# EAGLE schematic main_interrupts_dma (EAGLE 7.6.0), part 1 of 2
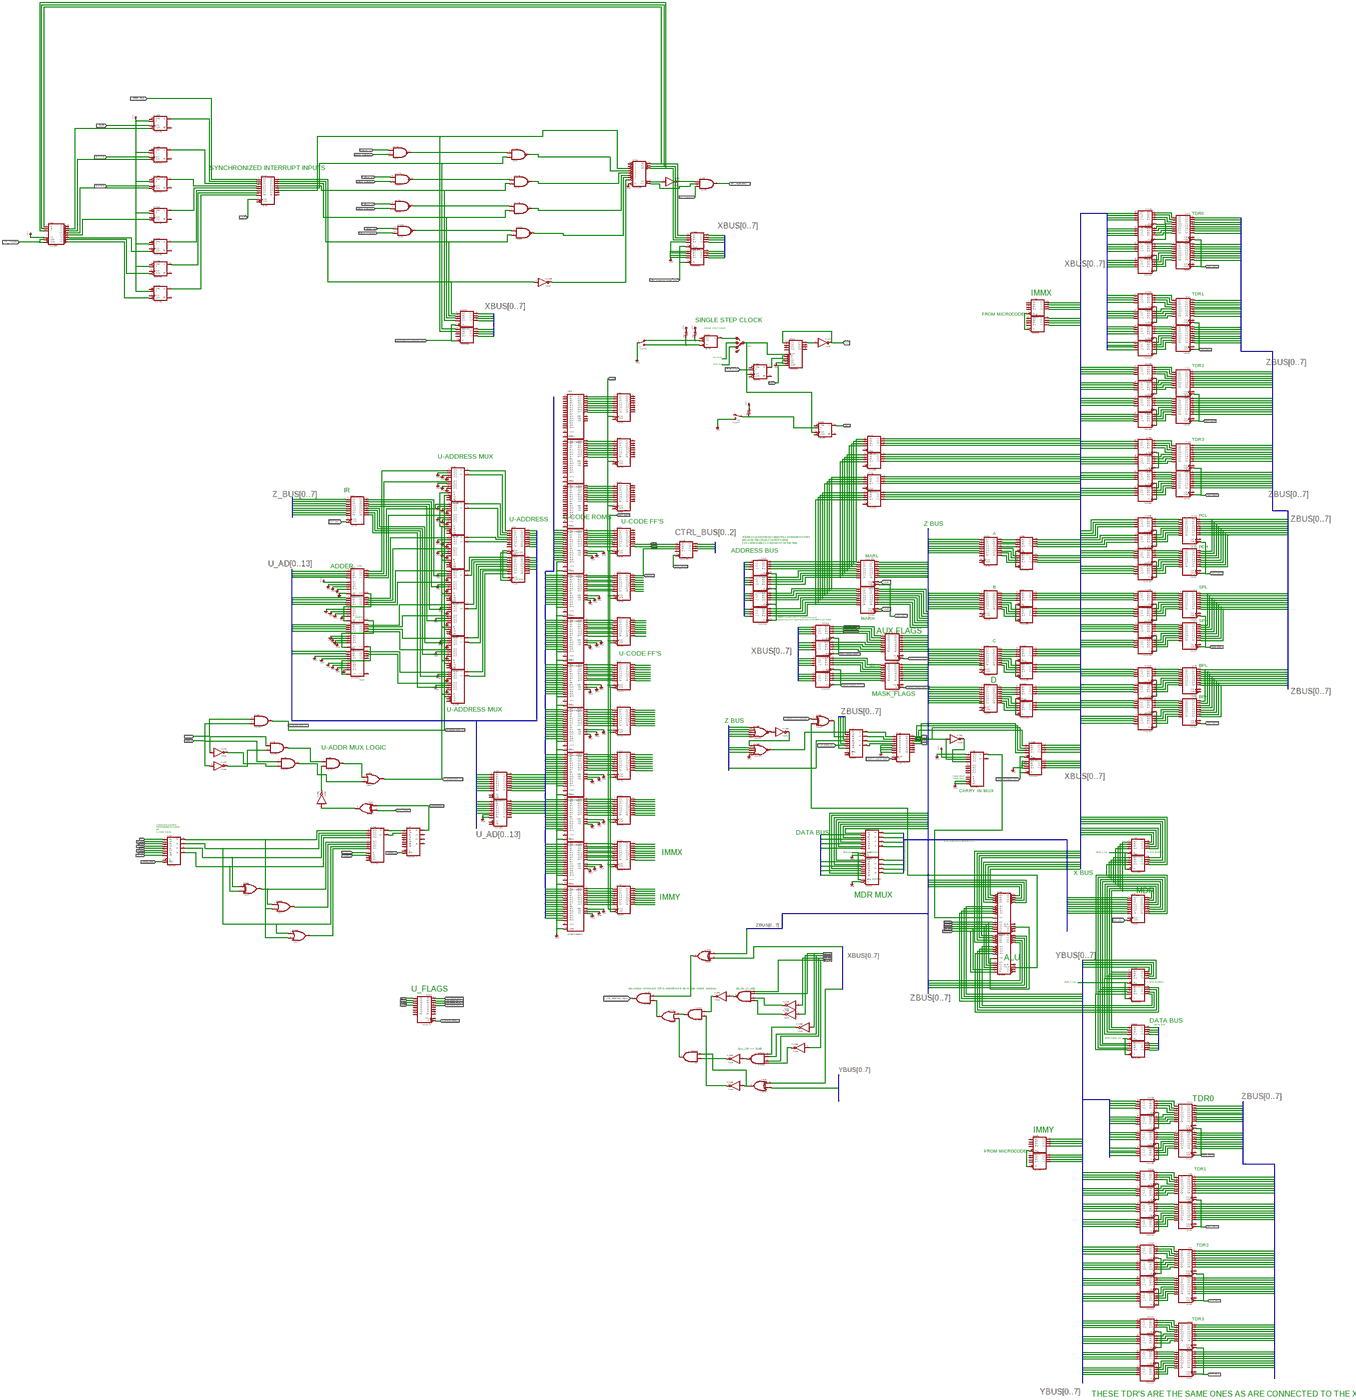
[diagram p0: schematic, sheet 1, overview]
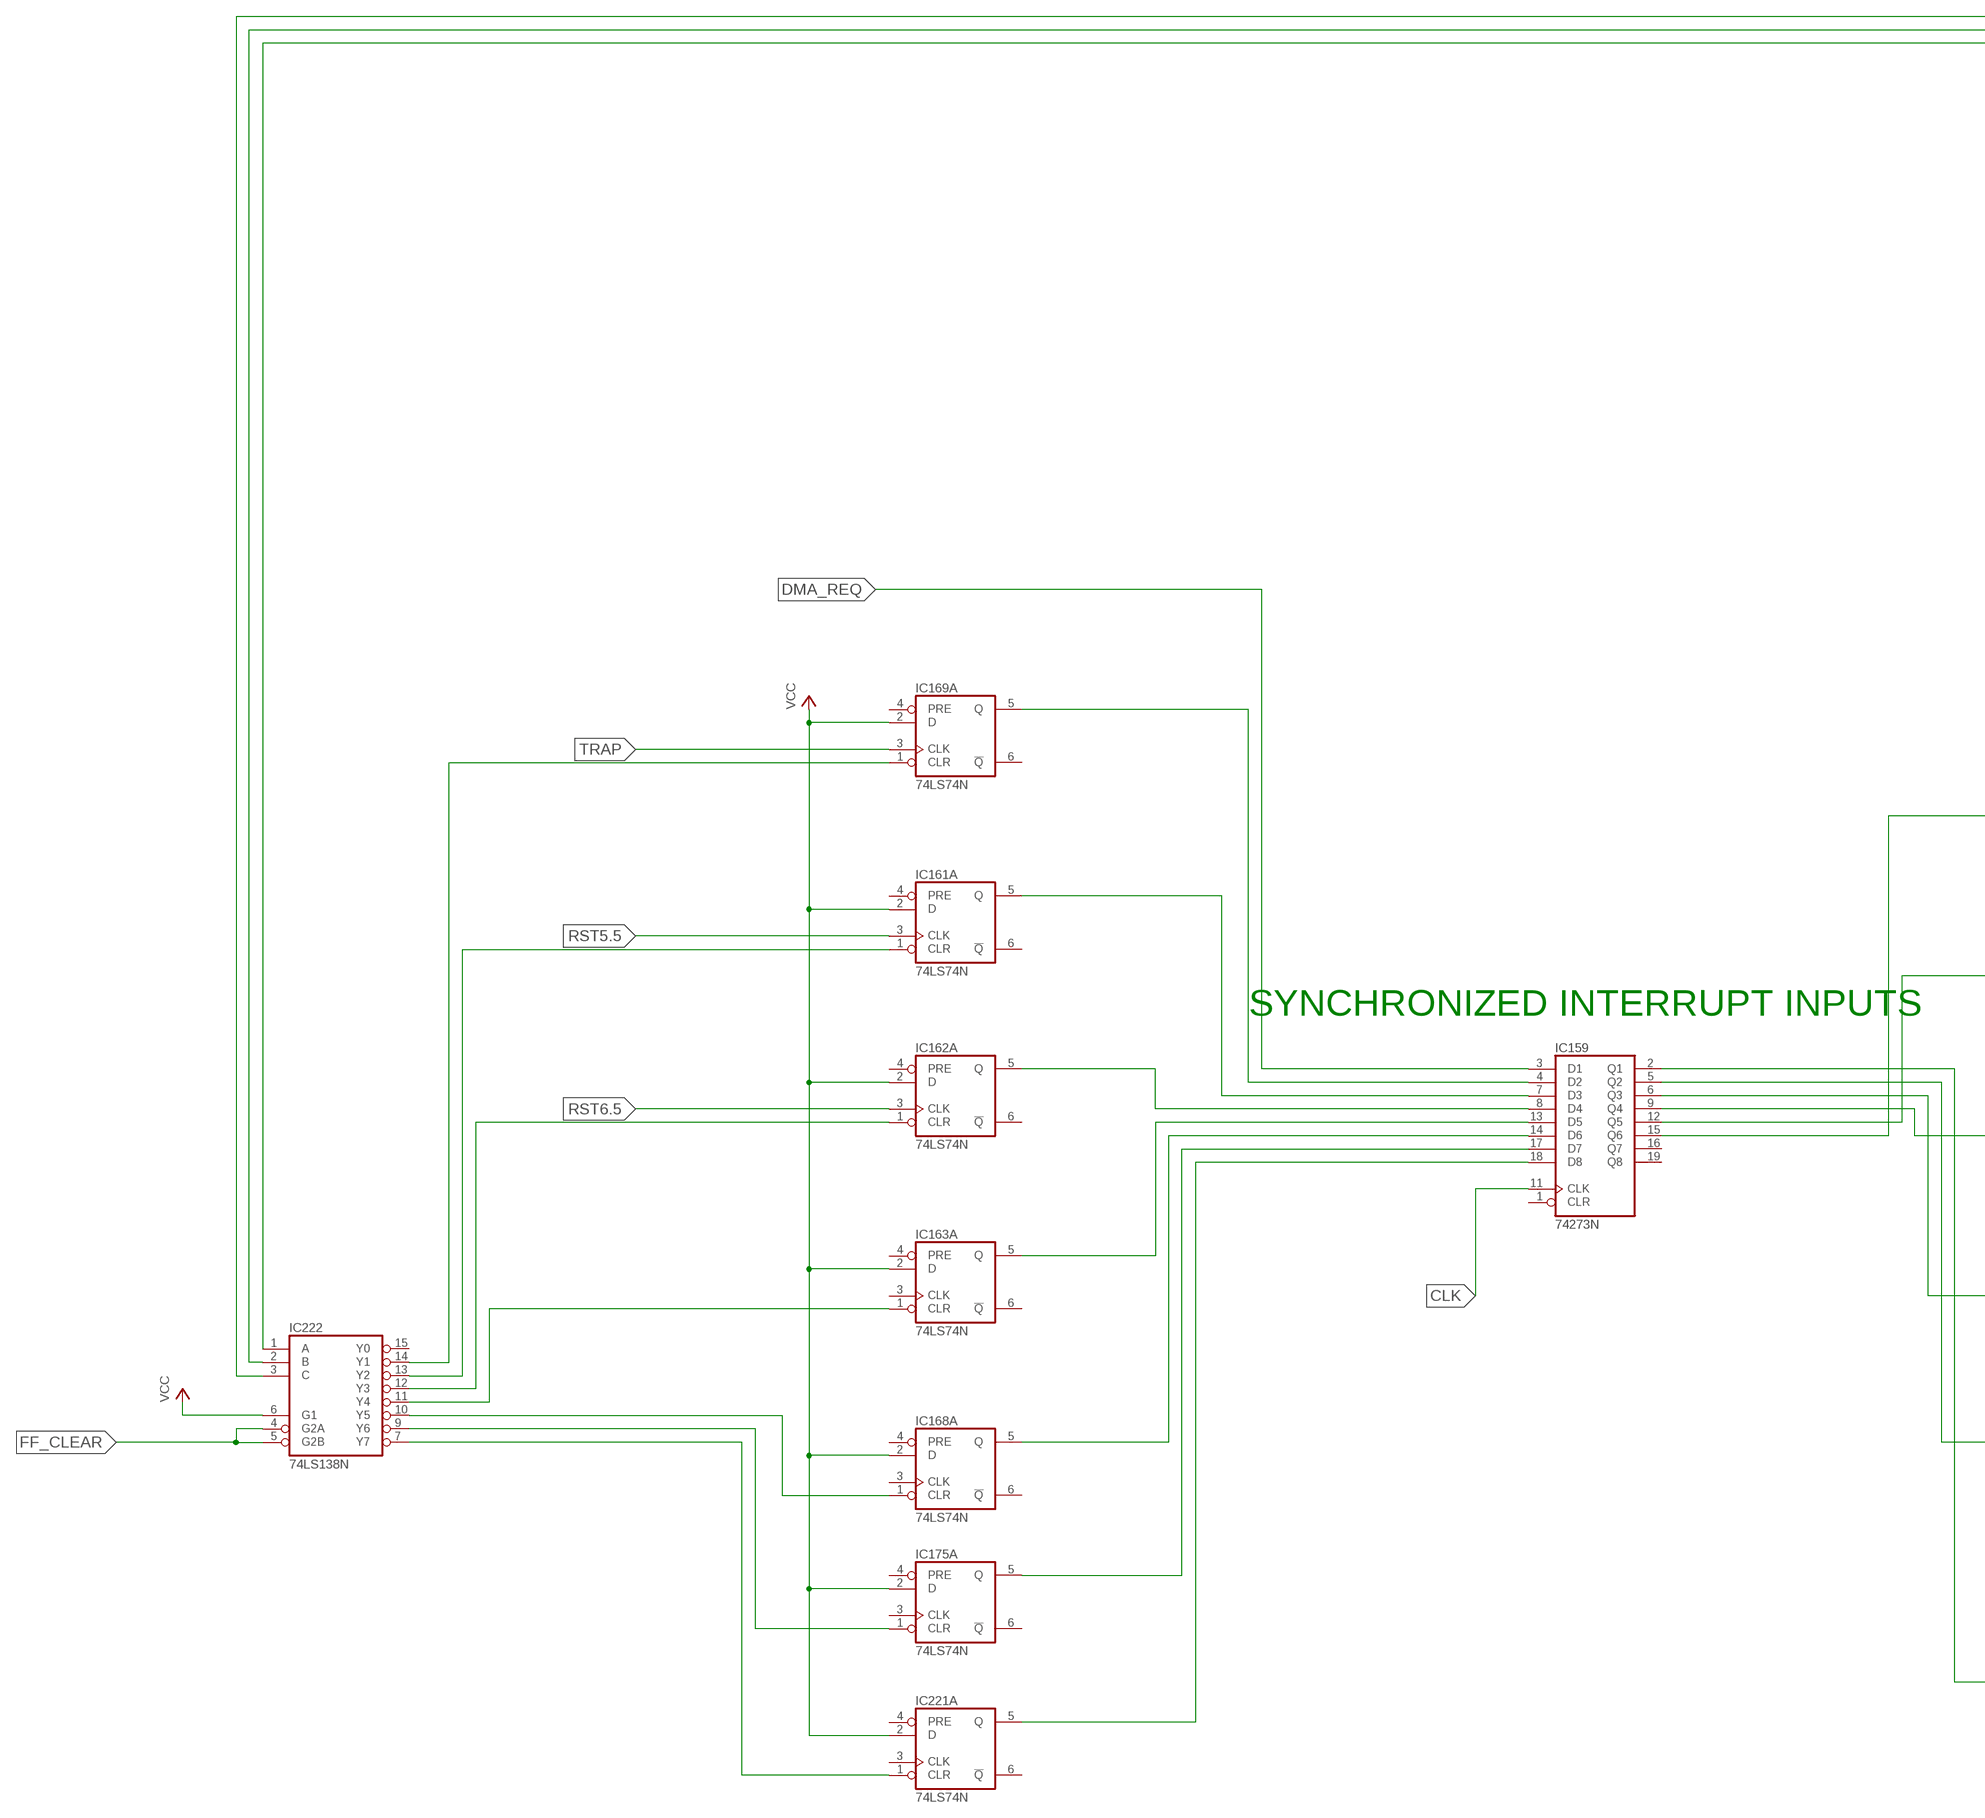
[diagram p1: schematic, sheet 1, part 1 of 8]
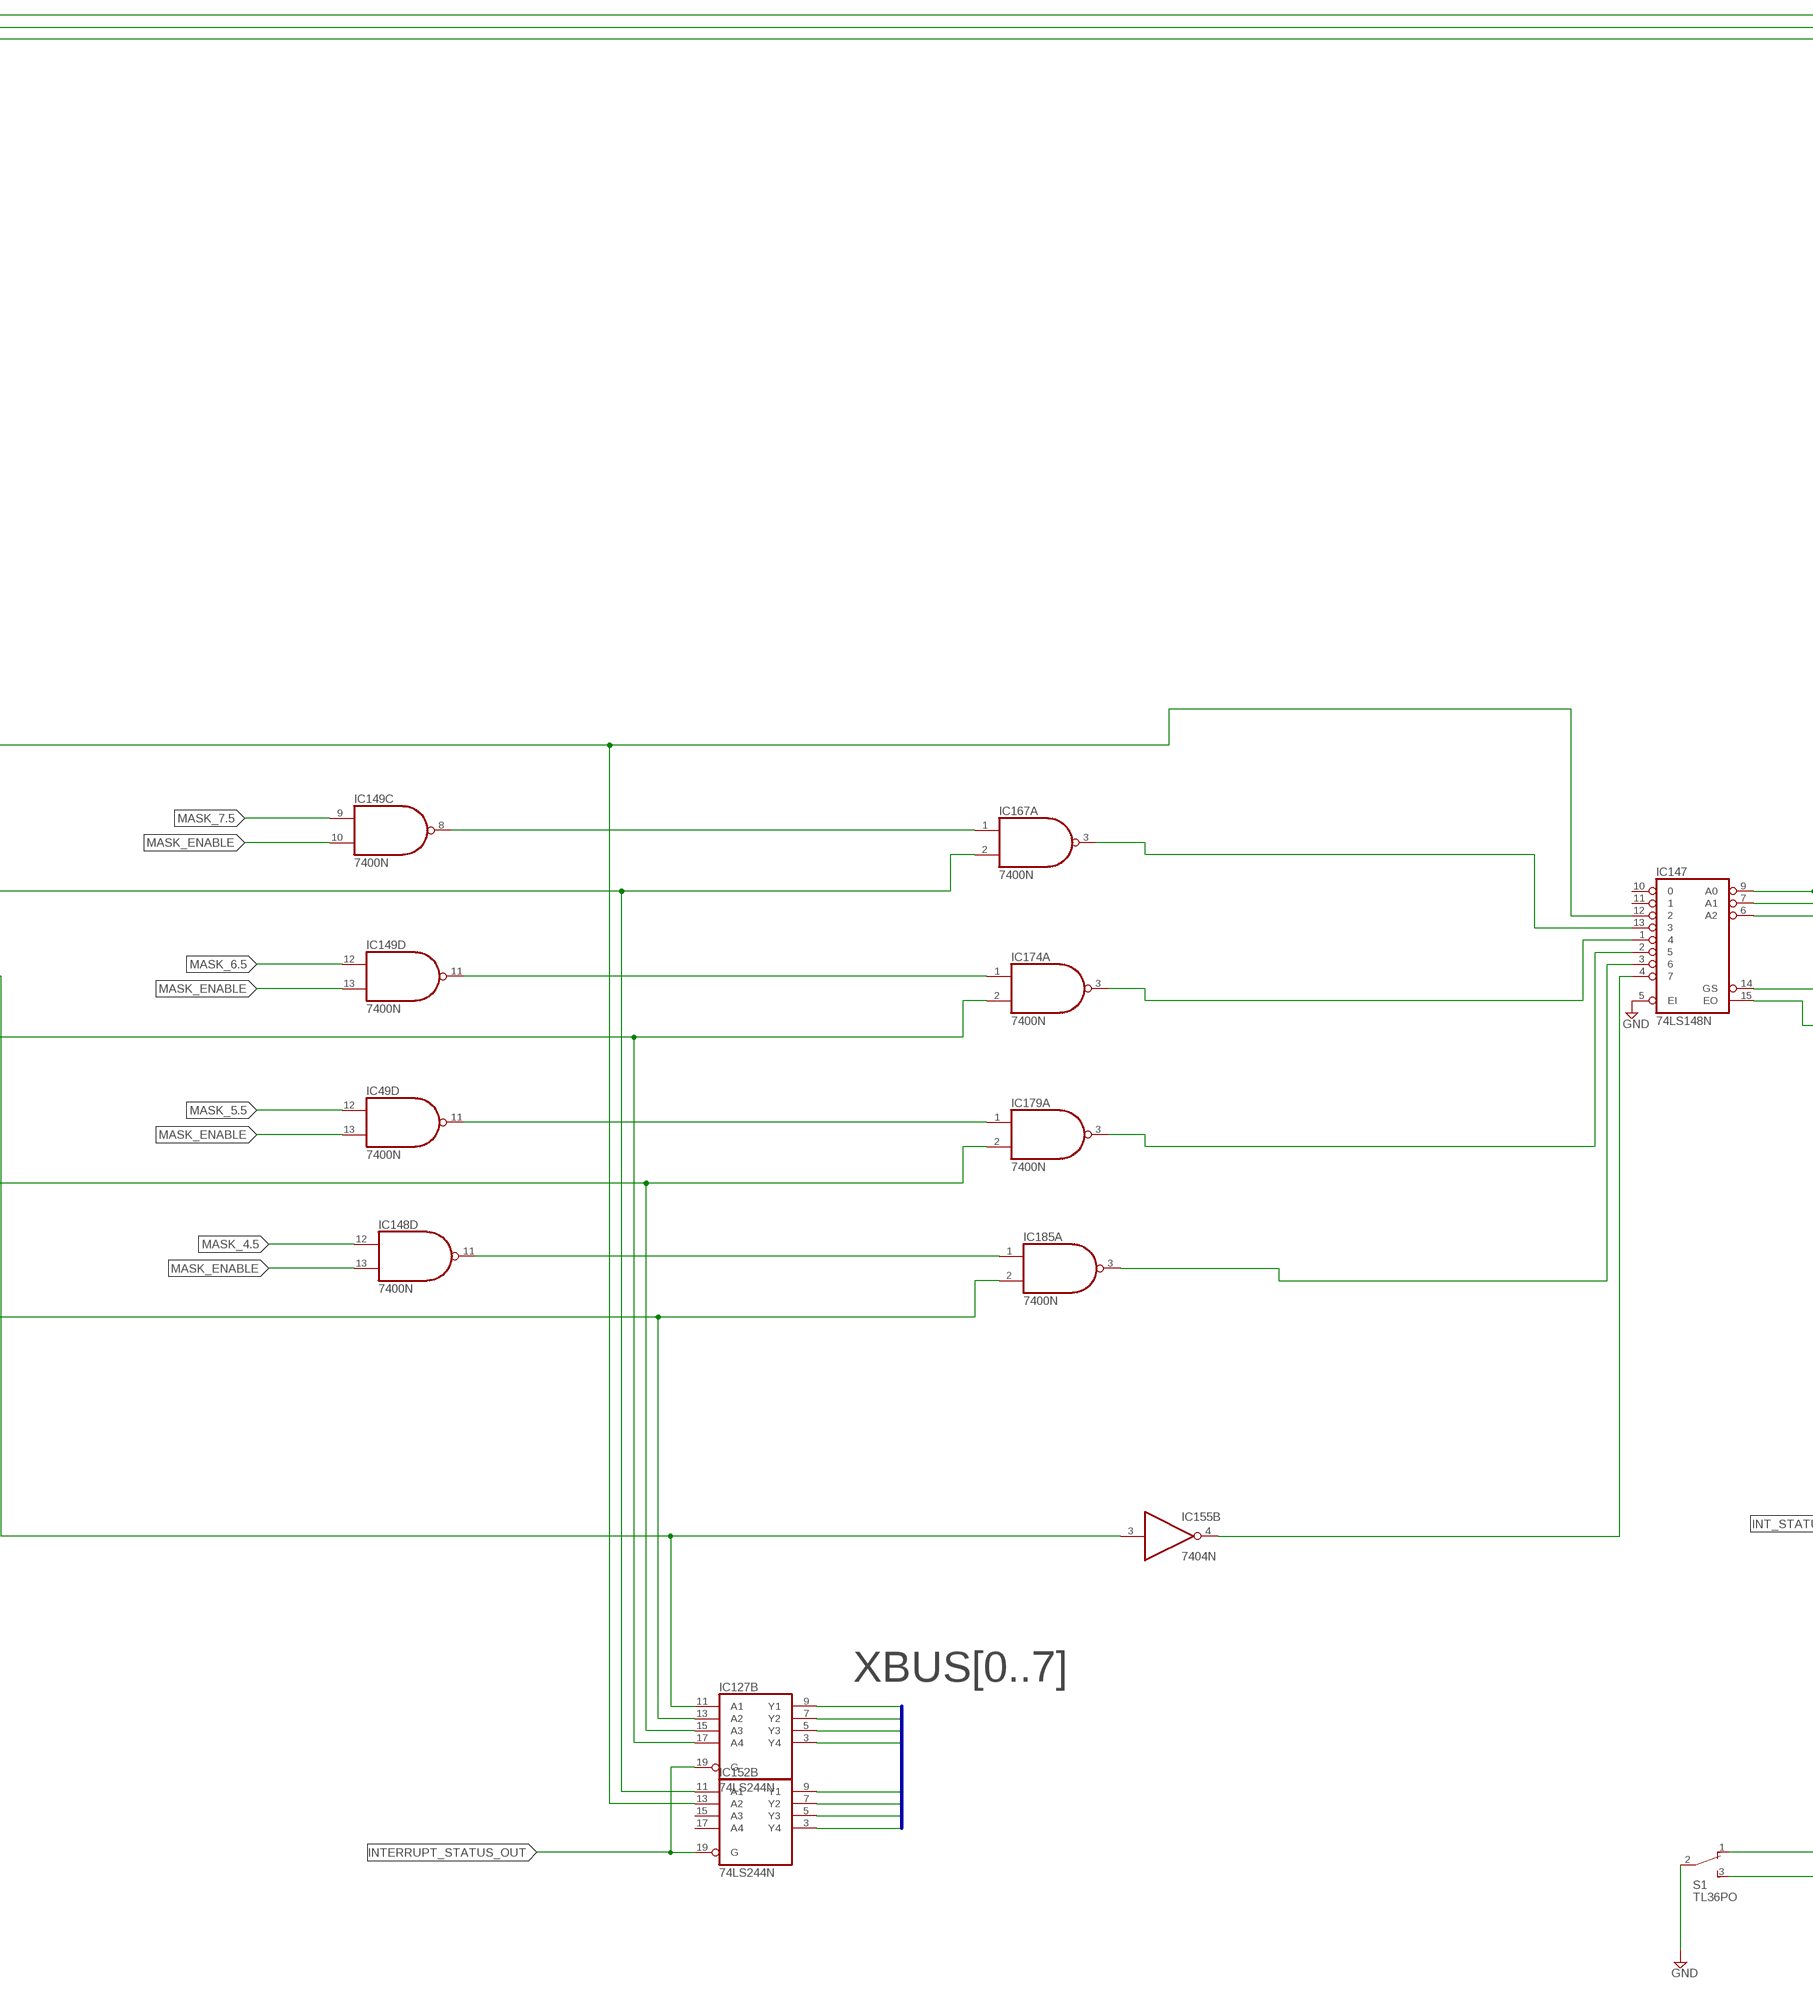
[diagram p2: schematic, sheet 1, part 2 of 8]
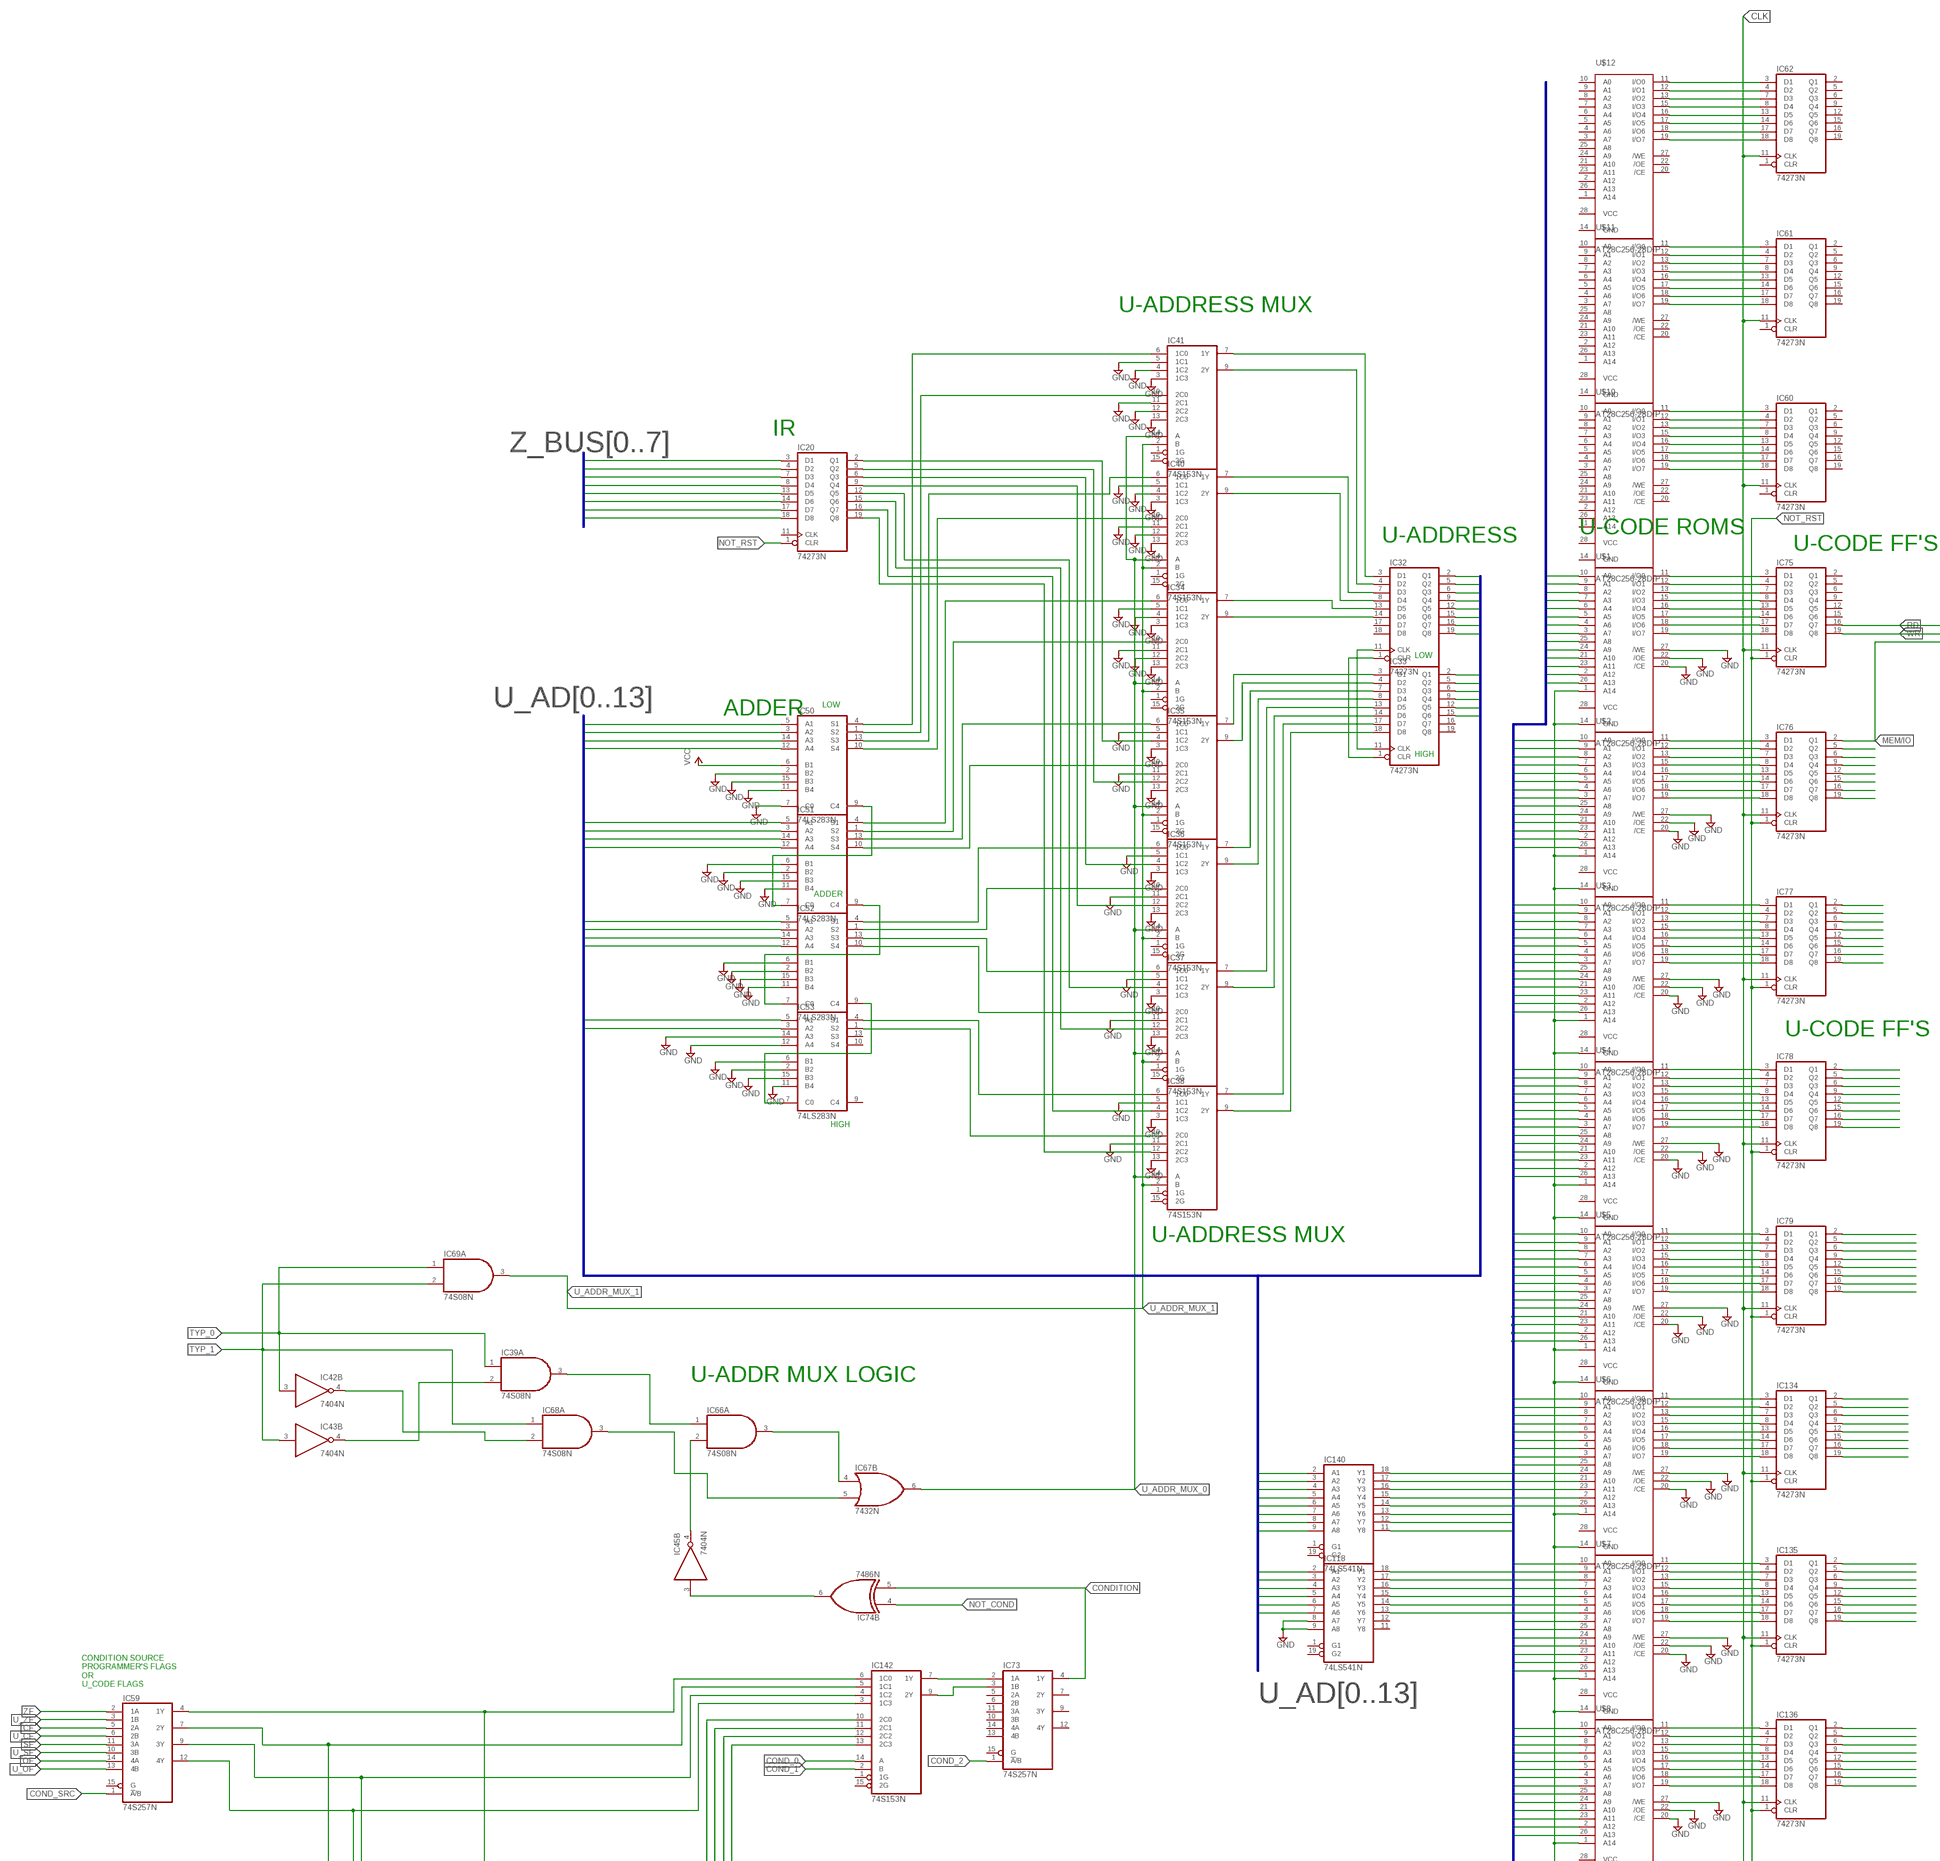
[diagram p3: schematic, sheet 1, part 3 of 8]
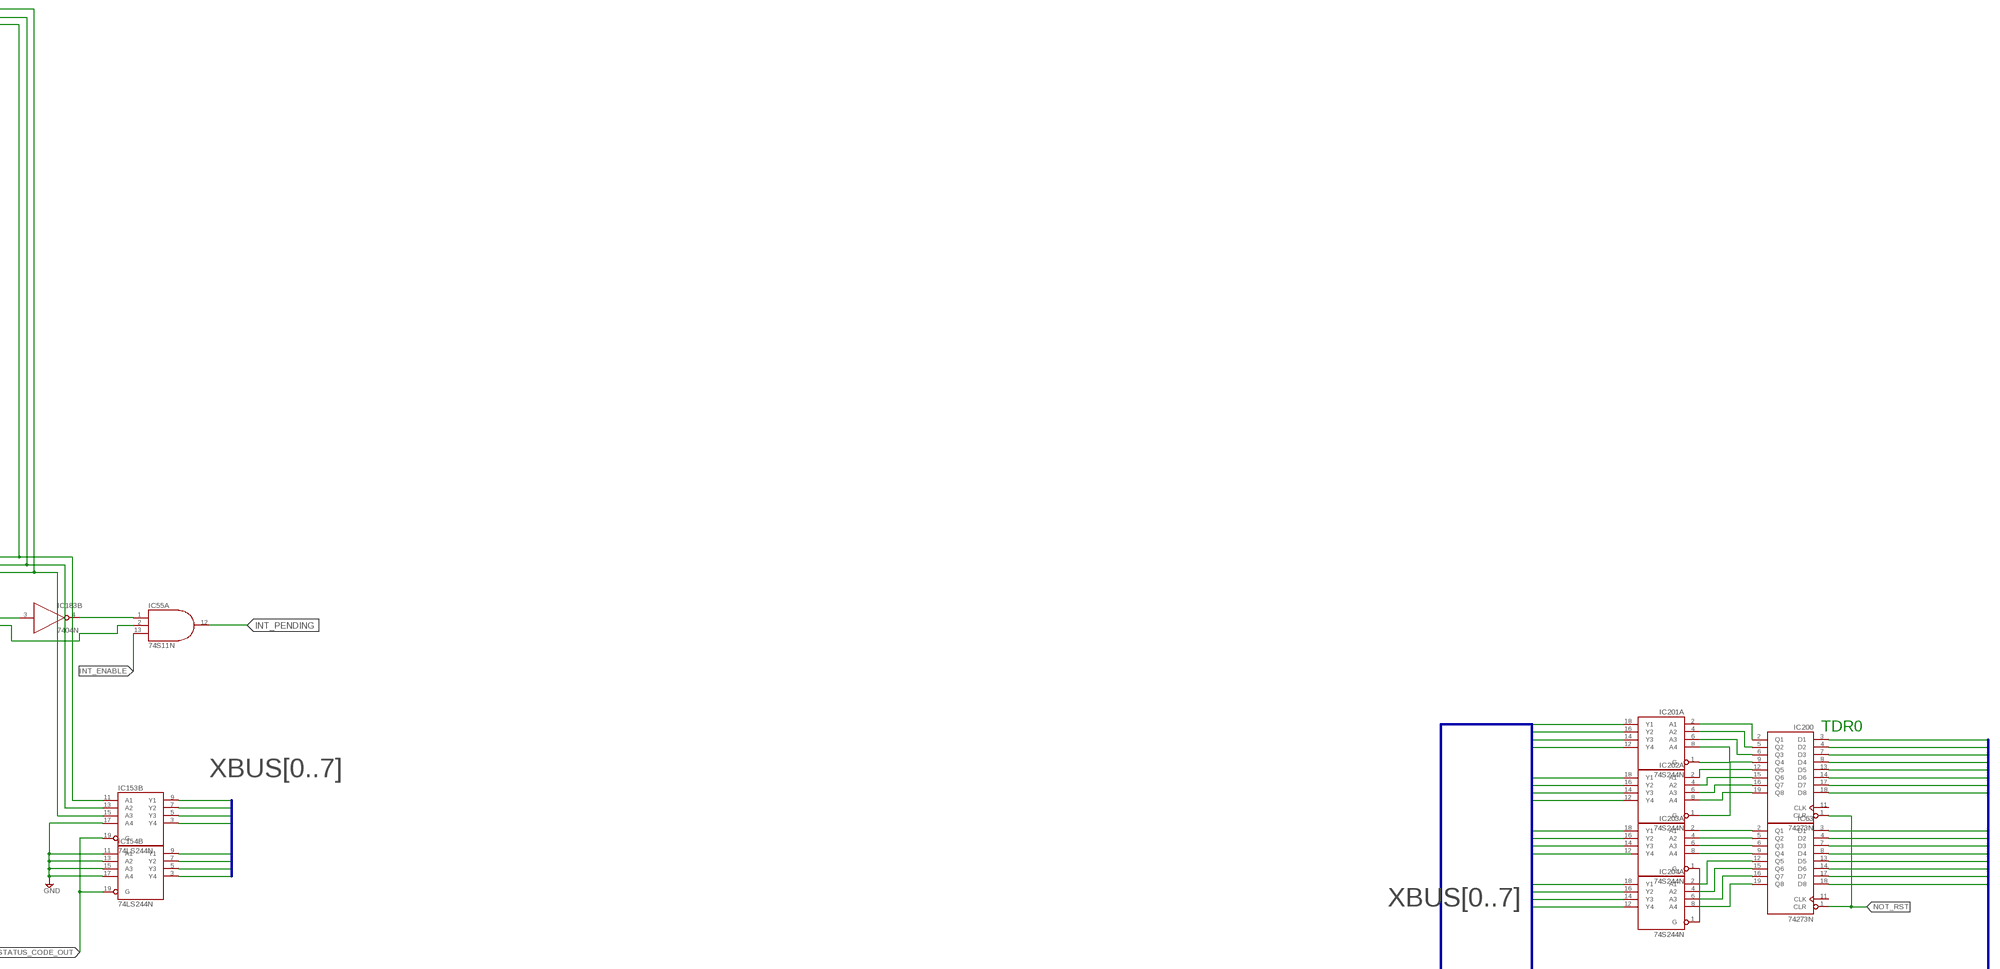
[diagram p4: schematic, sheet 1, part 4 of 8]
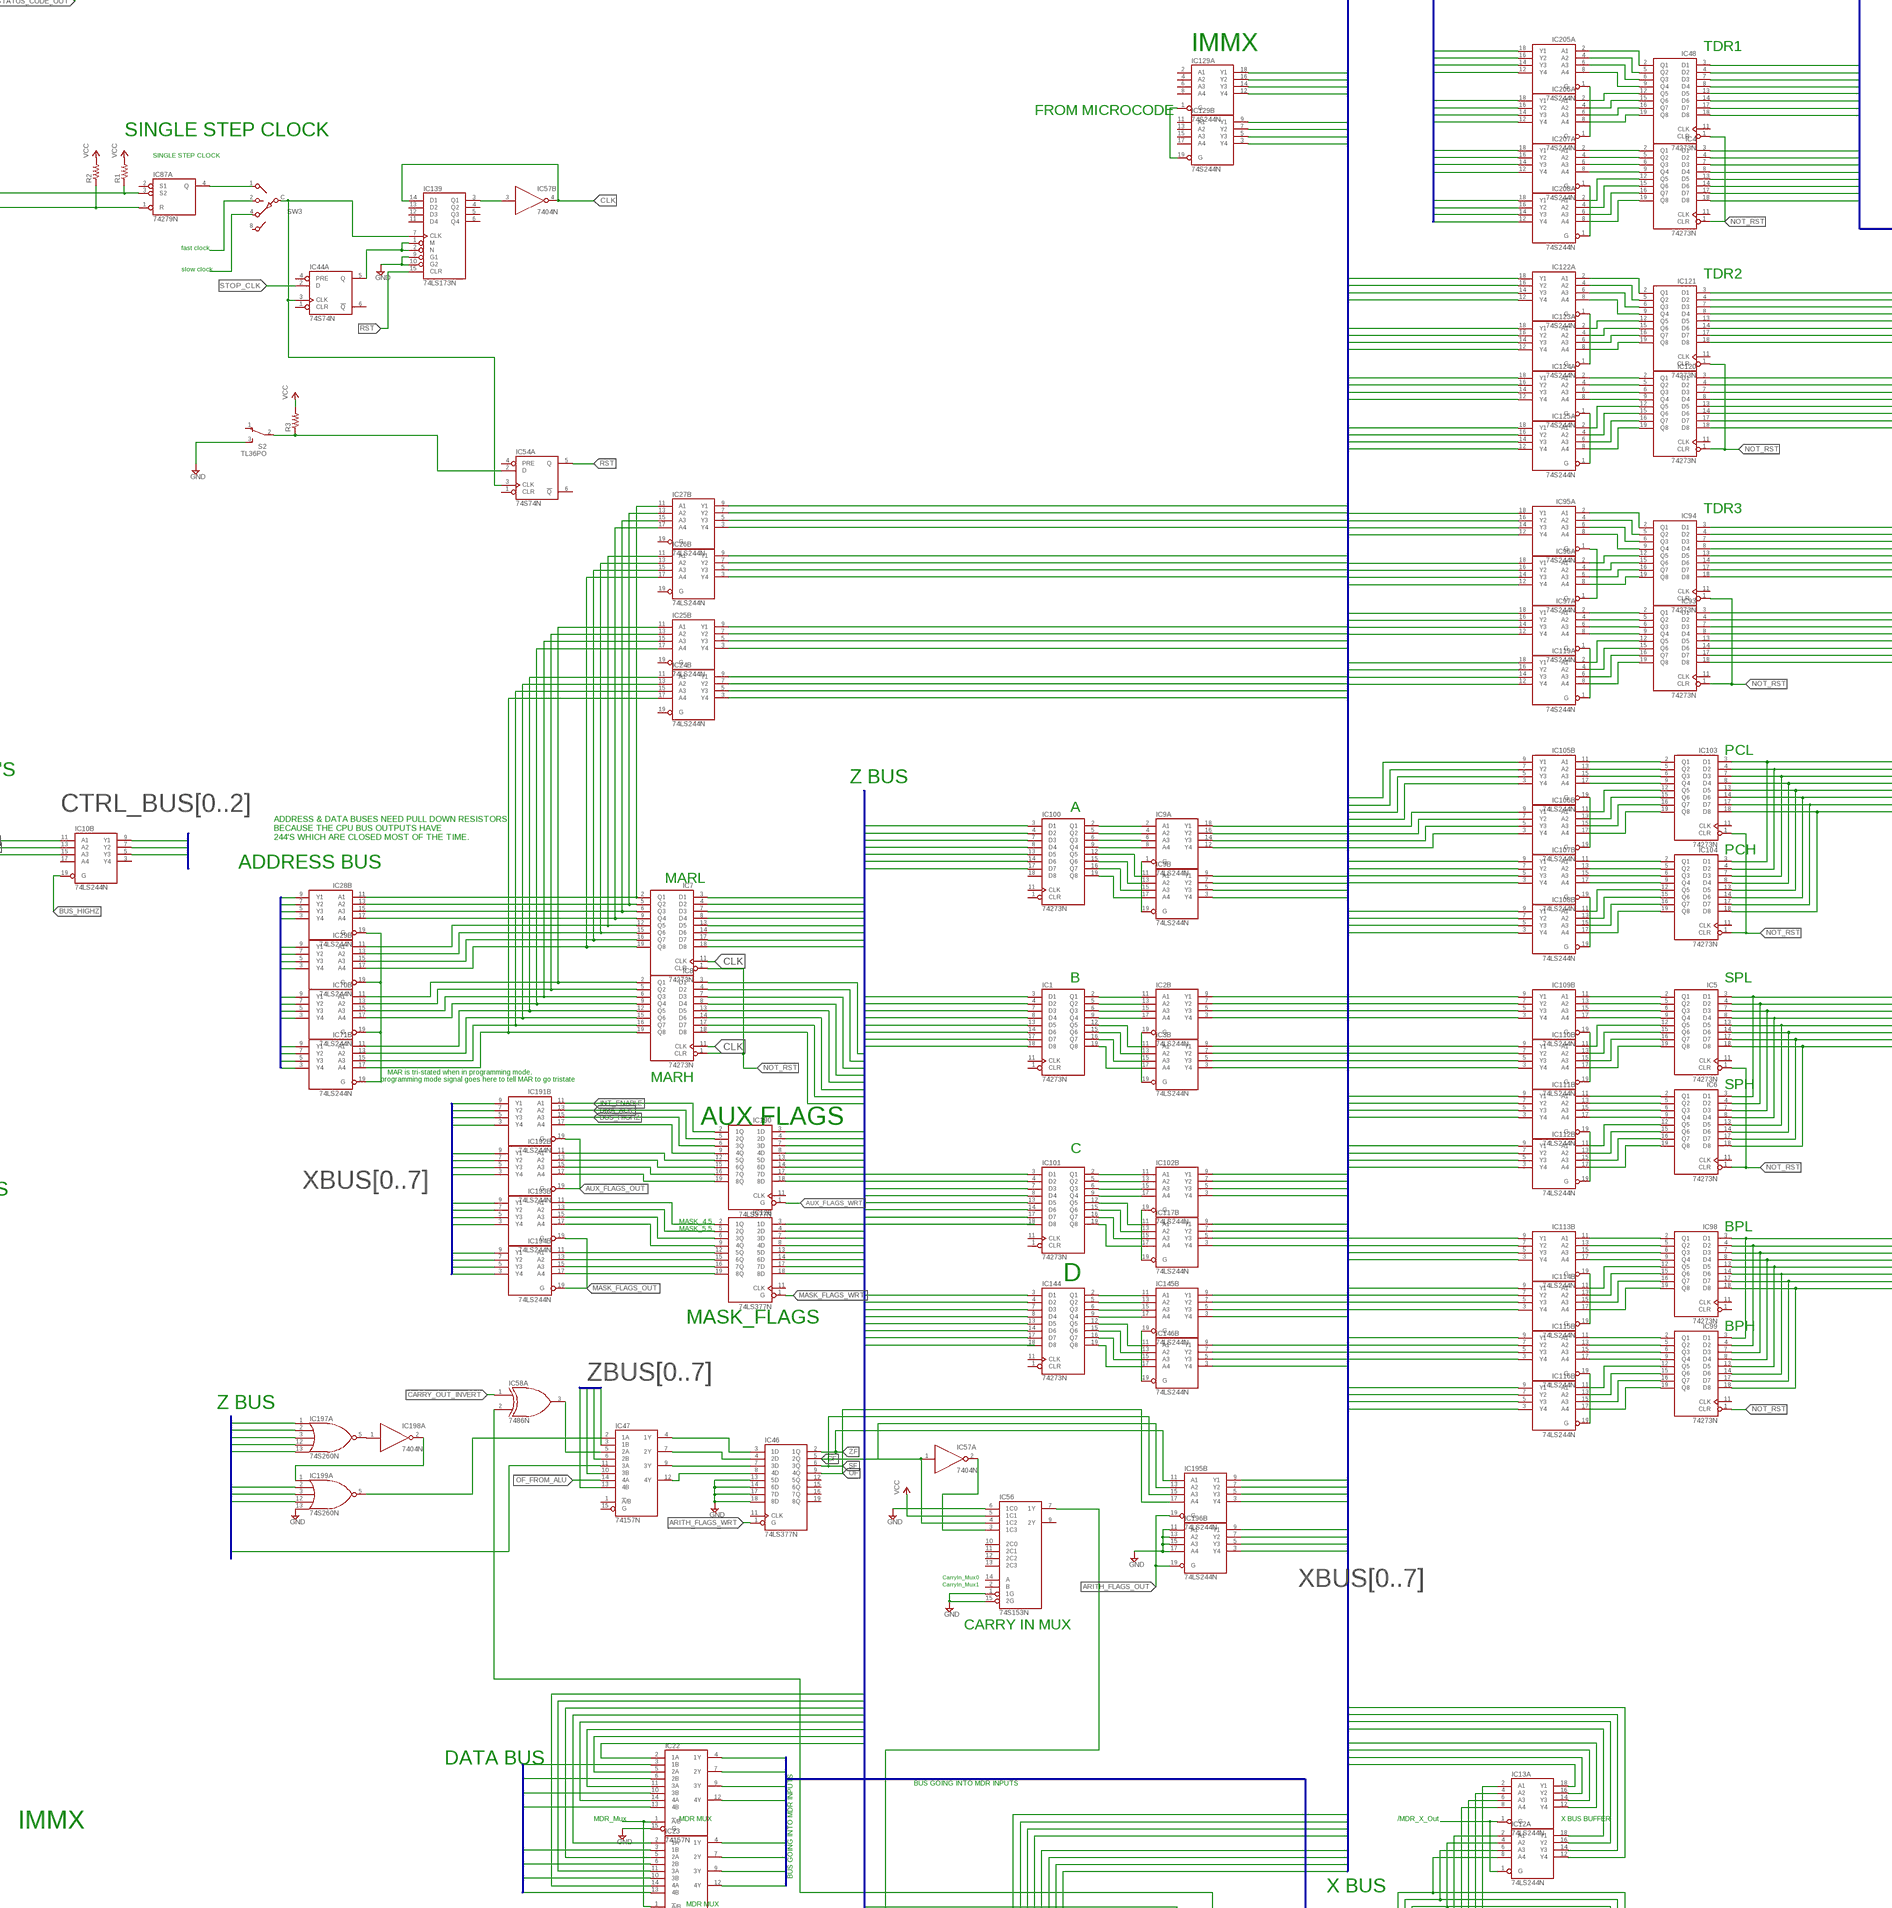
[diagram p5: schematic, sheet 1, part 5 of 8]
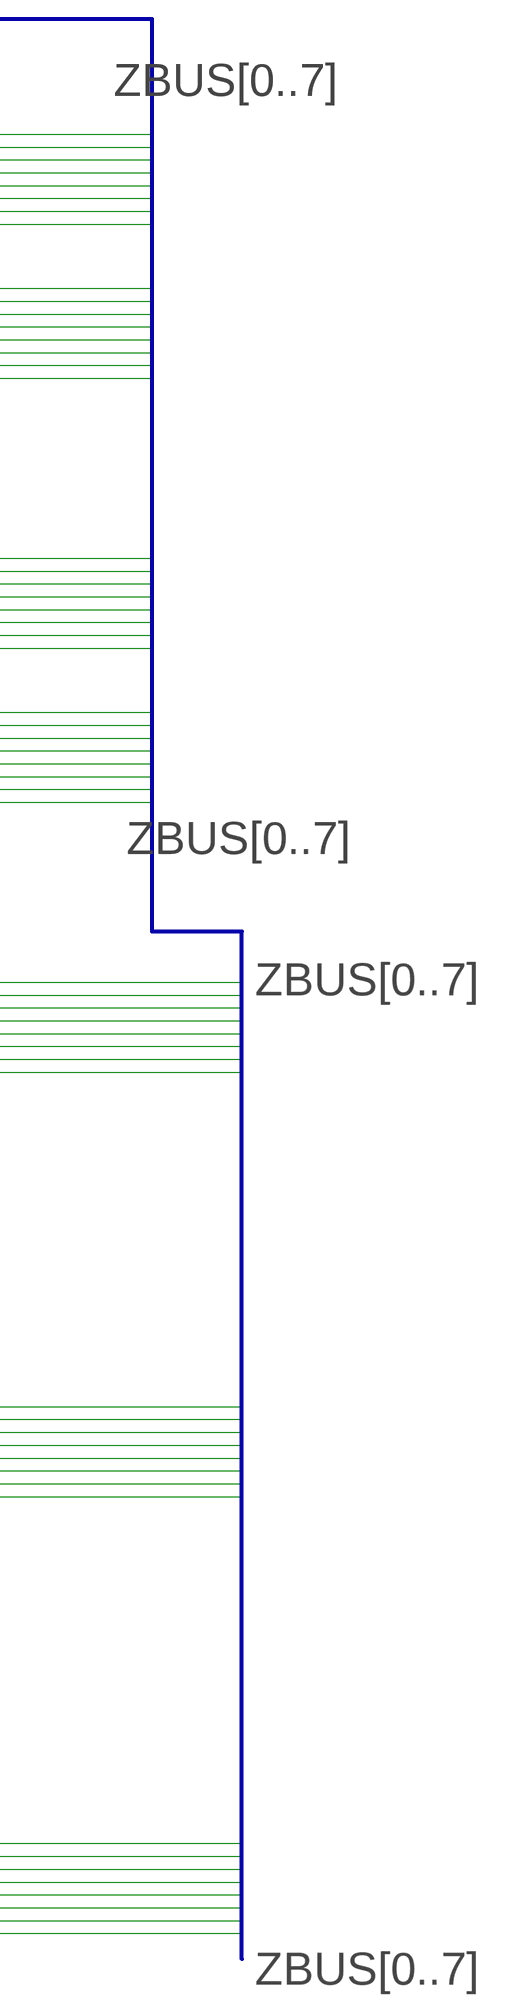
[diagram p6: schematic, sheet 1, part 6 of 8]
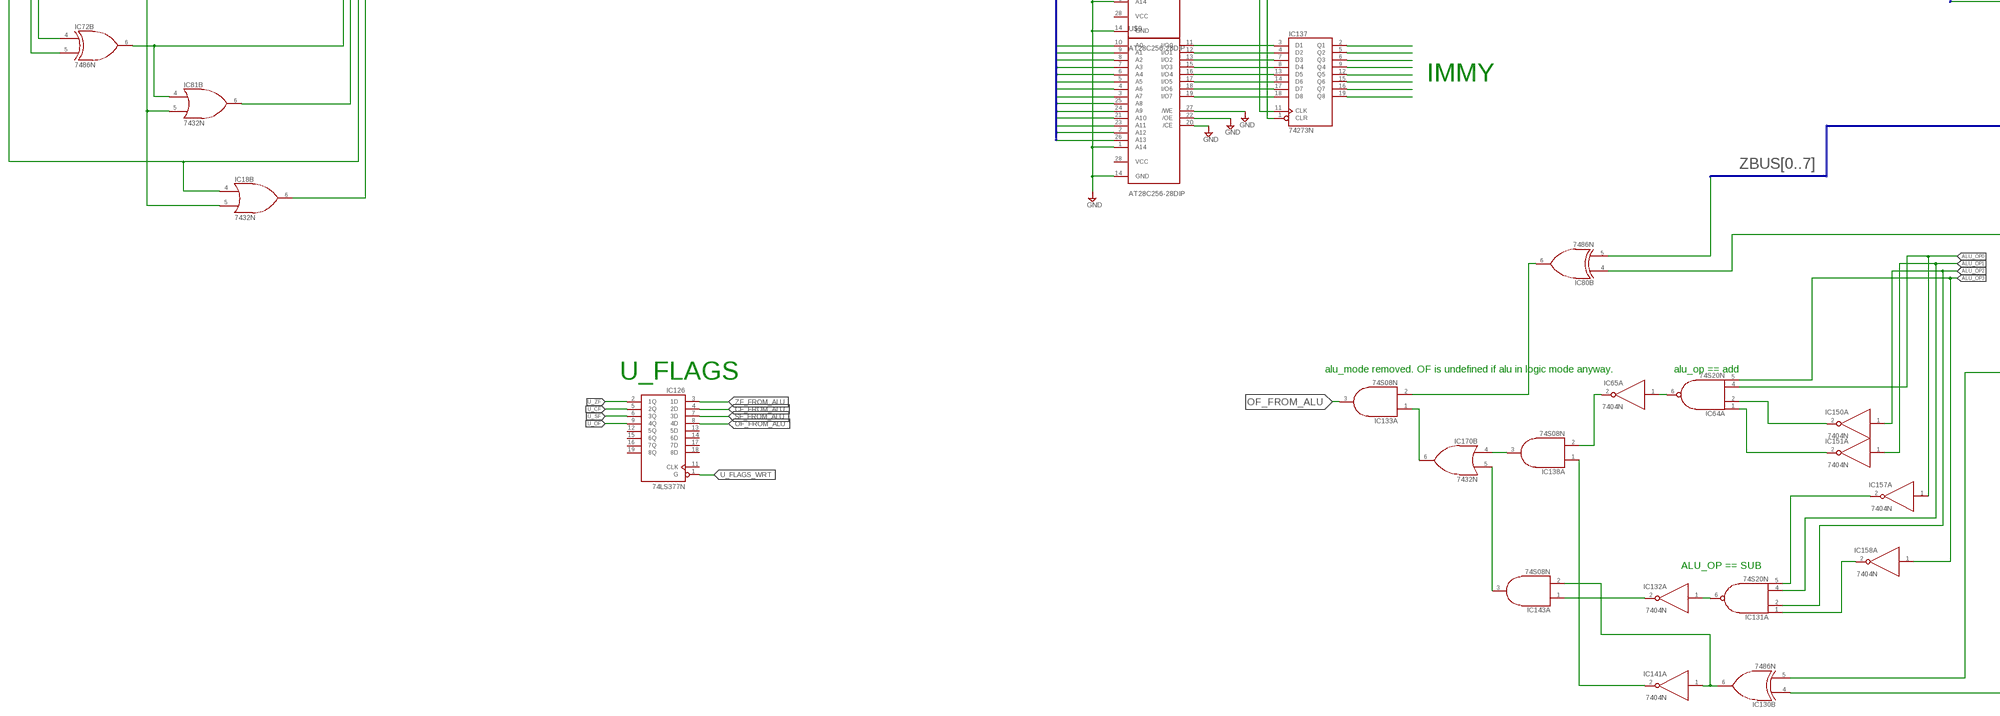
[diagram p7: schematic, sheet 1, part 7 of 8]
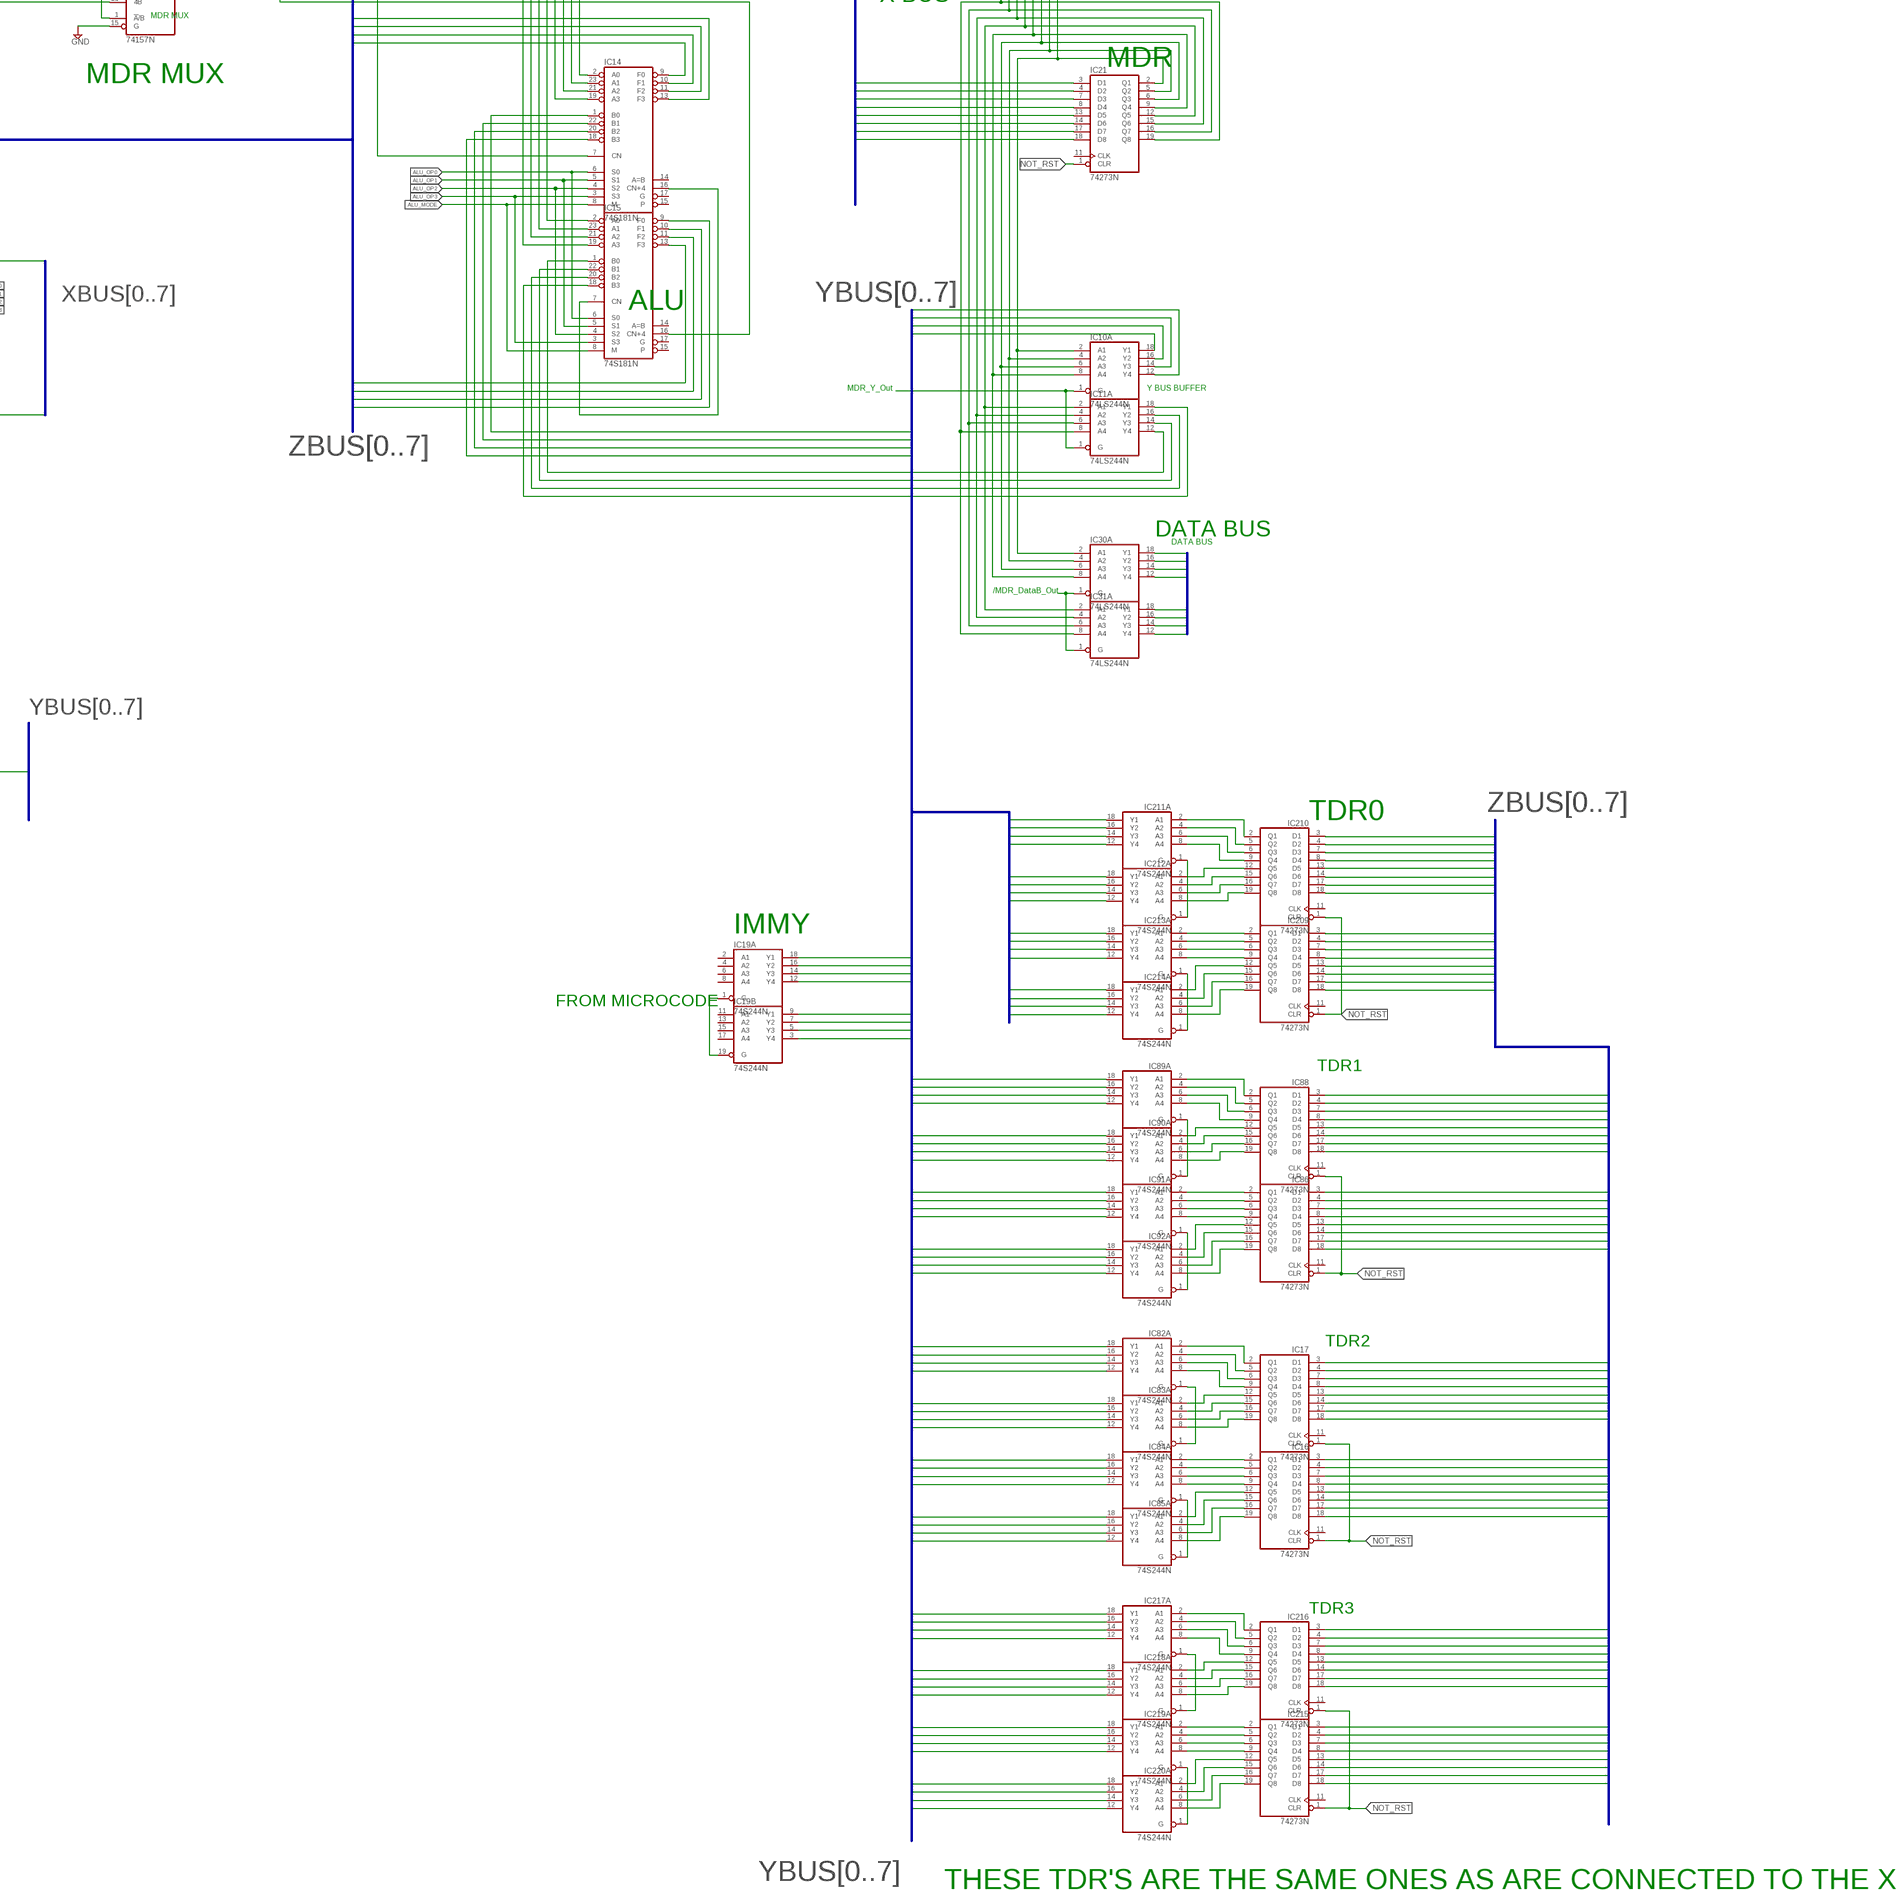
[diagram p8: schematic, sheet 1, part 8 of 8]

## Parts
IC1  74273N  [DIL20]
IC2  74LS244N  [DIL20]
IC3  74LS244N  [DIL20]
IC4  74273N  [DIL20]
IC5  74273N  [DIL20]
IC6  74273N  [DIL20]
IC7  74273N  [DIL20]
IC8  74273N  [DIL20]
IC9  74LS244N  [DIL20]
IC10  74LS244N  [DIL20]
IC11  74LS244N  [DIL20]
IC12  74LS244N  [DIL20]
IC13  74LS244N  [DIL20]
IC14  74S181N  [DIL24-6]
IC15  74S181N  [DIL24-6]
IC16  74273N  [DIL20]
IC17  74273N  [DIL20]
IC18  7432N  [DIL14]
IC19  74S244N  [DIL20]
IC20  74273N  [DIL20]
IC21  74273N  [DIL20]
IC22  74157N  [DIL16]
IC23  74157N  [DIL16]
IC24  74LS244N  [DIL20]
IC25  74LS244N  [DIL20]
IC26  74LS244N  [DIL20]
IC27  74LS244N  [DIL20]
IC28  74LS244N  [DIL20]
IC29  74LS244N  [DIL20]
IC30  74LS244N  [DIL20]
IC31  74LS244N  [DIL20]
IC32  74273N  [DIL20]
IC33  74273N  [DIL20]
IC34  74S153N  [DIL16]
IC35  74S153N  [DIL16]
IC36  74S153N  [DIL16]
IC37  74S153N  [DIL16]
IC38  74S153N  [DIL16]
IC39  74S08N  [DIL14]
IC40  74S153N  [DIL16]
IC41  74S153N  [DIL16]
IC42  7404N  [DIL14]
IC43  7404N  [DIL14]
IC44  74S74N  [DIL14]
IC45  7404N  [DIL14]
IC46  74LS377N  [DIL20]
IC47  74157N  [DIL16]
IC48  74273N  [DIL20]
IC49  7400N  [DIL14]
IC50  74LS283N  [DIL16]
IC51  74LS283N  [DIL16]
IC52  74LS283N  [DIL16]
IC53  74LS283N  [DIL16]
IC54  74S74N  [DIL14]
IC55  74S11N  [DIL14]
IC56  74S153N  [DIL16]
IC57  7404N  [DIL14]
IC58  7486N  [DIL14]
IC59  74S257N  [DIL16]
IC60  74273N  [DIL20]
IC61  74273N  [DIL20]
IC62  74273N  [DIL20]
IC63  74273N  [DIL20]
IC64  74S20N  [DIL14]
IC65  7404N  [DIL14]
IC66  74S08N  [DIL14]
IC67  7432N  [DIL14]
IC68  74S08N  [DIL14]
IC69  74S08N  [DIL14]
IC70  74LS244N  [DIL20]
IC71  74LS244N  [DIL20]
IC72  7486N  [DIL14]
IC73  74S257N  [DIL16]
IC74  7486N  [DIL14]
IC75  74273N  [DIL20]
IC76  74273N  [DIL20]
IC77  74273N  [DIL20]
IC78  74273N  [DIL20]
IC79  74273N  [DIL20]
IC80  7486N  [DIL14]
IC81  7432N  [DIL14]
IC82  74S244N  [DIL20]
IC83  74S244N  [DIL20]
IC84  74S244N  [DIL20]
IC85  74S244N  [DIL20]
IC86  74273N  [DIL20]
IC87  74279N  [DIL16]
IC88  74273N  [DIL20]
IC89  74S244N  [DIL20]
IC90  74S244N  [DIL20]
IC91  74S244N  [DIL20]
IC92  74S244N  [DIL20]
IC93  74273N  [DIL20]
IC94  74273N  [DIL20]
IC95  74S244N  [DIL20]
IC96  74S244N  [DIL20]
IC97  74S244N  [DIL20]
IC98  74273N  [DIL20]
IC99  74273N  [DIL20]
IC100  74273N  [DIL20]
IC101  74273N  [DIL20]
IC102  74LS244N  [DIL20]
IC103  74273N  [DIL20]
IC104  74273N  [DIL20]
IC105  74LS244N  [DIL20]
IC106  74LS244N  [DIL20]
IC107  74LS244N  [DIL20]
IC108  74LS244N  [DIL20]
IC109  74LS244N  [DIL20]
IC110  74LS244N  [DIL20]
IC111  74LS244N  [DIL20]
IC112  74LS244N  [DIL20]
IC113  74LS244N  [DIL20]
IC114  74LS244N  [DIL20]
IC115  74LS244N  [DIL20]
IC116  74LS244N  [DIL20]
IC117  74LS244N  [DIL20]
IC118  74LS541N  [DIL20]
IC119  74S244N  [DIL20]
IC120  74273N  [DIL20]
IC121  74273N  [DIL20]
IC122  74S244N  [DIL20]
IC123  74S244N  [DIL20]
IC124  74S244N  [DIL20]
IC125  74S244N  [DIL20]
IC126  74LS377N  [DIL20]
IC127  74LS244N  [DIL20]
IC128  74LS377N  [DIL20]
IC129  74S244N  [DIL20]
IC130  7486N  [DIL14]
IC131  74S20N  [DIL14]
IC132  7404N  [DIL14]
IC133  74S08N  [DIL14]
IC134  74273N  [DIL20]
IC135  74273N  [DIL20]
IC136  74273N  [DIL20]
IC137  74273N  [DIL20]
IC138  74S08N  [DIL14]
IC139  74LS173N  [DIL16]
IC140  74LS541N  [DIL20]
IC141  7404N  [DIL14]
IC142  74S153N  [DIL16]
IC143  74S08N  [DIL14]
IC144  74273N  [DIL20]
IC145  74LS244N  [DIL20]
IC146  74LS244N  [DIL20]
IC147  74LS148N  [DIL16]
IC148  7400N  [DIL14]
IC149  7400N  [DIL14]
IC150  7404N  [DIL14]
IC151  7404N  [DIL14]
IC152  74LS244N  [DIL20]
IC153  74LS244N  [DIL20]
IC154  74LS244N  [DIL20]
IC155  7404N  [DIL14]
IC157  7404N  [DIL14]
IC158  7404N  [DIL14]
IC159  74273N  [DIL20]
IC161  74LS74N  [DIL14]
IC162  74LS74N  [DIL14]
IC163  74LS74N  [DIL14]
IC167  7400N  [DIL14]
IC168  74LS74N  [DIL14]
IC169  74LS74N  [DIL14]
IC170  7432N  [DIL14]
IC174  7400N  [DIL14]
IC175  74LS74N  [DIL14]
IC179  7400N  [DIL14]
IC183  7404N  [DIL14]
IC185  7400N  [DIL14]
IC190  74LS377N  [DIL20]
IC191  74LS244N  [DIL20]
IC192  74LS244N  [DIL20]
IC193  74LS244N  [DIL20]
IC194  74LS244N  [DIL20]
IC195  74LS244N  [DIL20]
IC196  74LS244N  [DIL20]
IC197  74S260N  [DIL14]
IC198  7404N  [DIL14]
IC199  74S260N  [DIL14]
IC200  74273N  [DIL20]
IC201  74S244N  [DIL20]
IC202  74S244N  [DIL20]
IC203  74S244N  [DIL20]
IC204  74S244N  [DIL20]
IC205  74S244N  [DIL20]
IC206  74S244N  [DIL20]
IC207  74S244N  [DIL20]
IC208  74S244N  [DIL20]
IC209  74273N  [DIL20]
IC210  74273N  [DIL20]
IC211  74S244N  [DIL20]
IC212  74S244N  [DIL20]
IC213  74S244N  [DIL20]
IC214  74S244N  [DIL20]
IC215  74273N  [DIL20]
IC216  74273N  [DIL20]
IC217  74S244N  [DIL20]
IC218  74S244N  [DIL20]
IC219  74S244N  [DIL20]
IC220  74S244N  [DIL20]
IC221  74LS74N  [DIL14]
IC222  74LS138N  [DIL16]
R1  R-US_0204/2V  [0204V]
R2  R-US_0204/2V  [0204V]
R3  R-US_0204/2V  [0204V]
S1  TL36PO  [TL3XPO]
S2  TL36PO  [TL3XPO]
SW3  SW-C10  [SW-C10]
U$1  AT28C256-28DIP  [DIL28-6]
U$2  AT28C256-28DIP  [DIL28-6]
U$3  AT28C256-28DIP  [DIL28-6]
U$4  AT28C256-28DIP  [DIL28-6]
U$5  AT28C256-28DIP  [DIL28-6]
U$6  AT28C256-28DIP  [DIL28-6]
U$7  AT28C256-28DIP  [DIL28-6]
U$8  AT28C256-28DIP  [DIL28-6]
U$9  AT28C256-28DIP  [DIL28-6]
U$10  AT28C256-28DIP  [DIL28-6]
U$11  AT28C256-28DIP  [DIL28-6]
U$12  AT28C256-28DIP  [DIL28-6]

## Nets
45435: IC18.5(B:I1) IC59.4(1Y) IC81.5(B:I1) IC142.6(1C0)
345345: IC59.9(3Y) IC72.4(B:I0) IC142.4(1C2)
634354: IC18.4(B:I0) IC59.7(2Y) IC142.5(1C1) IC142.12(2C2)
4654654: IC59.12(4Y) IC72.5(B:I1) IC142.3(1C3)
AD0: IC28.9(B:Y1)
AD1: IC28.7(B:Y2)
AD2: IC28.5(B:Y3)
AD3: IC28.3(B:Y4)
AD4: IC29.9(B:Y1)
AD5: IC29.7(B:Y2)
AD6: IC29.5(B:Y3)
AD7: IC29.3(B:Y4)
AD8: IC70.9(B:Y1)
AD9: IC70.7(B:Y2)
AD10: IC70.5(B:Y3)
AD11: IC70.3(B:Y4)
AD12: IC71.9(B:Y1)
AD13: IC71.7(B:Y2)
AD14: IC71.5(B:Y3)
AD15: IC71.3(B:Y4)
ALU_MODE: IC14.8(M) IC15.8(M)
ALU_OP0: IC14.6(S0) IC15.6(S0) IC64.4(A:I2) IC157.1(A:I)
ALU_OP1: IC14.5(S1) IC15.5(S1) IC131.4(A:I2) IC151.1(A:I)
ALU_OP2: IC14.4(S2) IC15.4(S2) IC131.2(A:I1) IC150.1(A:I)
ALU_OP3: IC14.3(S3) IC15.3(S3) IC64.5(A:I3) IC158.1(A:I)
ARITH_FLAGS_OUT: IC195.19(B:G) IC196.19(B:G)
AUX_FLAGS_OUT: IC191.19(B:G) IC192.19(B:G)
AUX_FLAGS_WRT: IC190.1(G)
BUS_HIGHZ: IC10.19(B:G) IC28.19(B:G) IC29.19(B:G) IC70.19(B:G) IC71.19(B:G) IC190.6(3Q) IC191.15(B:A3)
CALL_RST_5.5: IC147.3 IC185.3(A:O)
CARRY_OUT_INVERT: IC58.1(A:I0)
CF: IC46.5(2Q) IC56.4(1C2) IC57.1(A:I) IC59.5(2A) IC195.13(B:A2)
CF_FROM_ALU: IC126.4(2D)
CLK: IC7.11(CLK) IC8.11(CLK) IC57.4(B:O) IC60.11(CLK) IC61.11(CLK) IC62.11(CLK) IC75.11(CLK) IC76.11(CLK) IC77.11(CLK) IC78.11(CLK) IC79.11(CLK) IC134.11(CLK) IC135.11(CLK) IC136.11(CLK) IC137.11(CLK) IC139.14(D1) IC159.11(CLK)
COND_0: IC142.14(A)
COND_1: IC142.2(B)
COND_2: IC73.1(!A!/B)
COND_SRC: IC59.1(!A!/B)
CONDITION: IC73.4(1Y) IC74.5(B:I1)
CTRL_BUS0: IC10.9(B:Y1)
CTRL_BUS1: IC10.7(B:Y2)
CTRL_BUS2: IC10.5(B:Y3)
DATA0: IC20.3(D1)
DATA1: IC20.4(D2)
DATA2: IC20.7(D3)
DATA3: IC20.8(D4)
DATA4: IC20.13(D5)
DATA5: IC20.14(D6)
DATA6: IC20.17(D7)
DATA7: IC20.18(D8)
DMA_ACK: IC190.5(2Q) IC191.13(B:A2)
DMA_REQ: IC127.11(B:A1) IC155.3(B:I) IC159.2(Q1) IC159.3(D1)
FF_CLEAR: IC222.4(G2A) IC222.5(G2B)
GND: IC22.15(G) IC23.15(G) IC34.3(1C3) IC34.4(1C2) IC34.5(1C1) IC34.11(2C1) IC34.12(2C2) IC34.13(2C3) IC35.3(1C3) IC35.5(1C1) IC35.11(2C1) IC35.13(2C3) IC36.3(1C3) IC36.5(1C1) IC36.11(2C1) IC36.13(2C3) IC37.3(1C3) IC37.5(1C1) IC37.11(2C1) IC37.13(2C3) IC38.3(1C3) IC38.5(1C1) IC38.11(2C1) IC38.13(2C3) IC40.3(1C3) IC40.4(1C2) IC40.5(1C1) IC40.11(2C1) IC40.12(2C2) IC40.13(2C3) IC41.3(1C3) IC41.4(1C2) IC41.5(1C1) IC41.11(2C1) IC41.12(2C2) IC41.13(2C3) IC46.13(5D) IC46.14(6D) IC46.17(7D) IC46.18(8D) IC50.2(B2) IC50.7(C0) IC50.11(B4) IC50.15(B3) IC51.2(B2) IC51.6(B1) IC51.11(B4) IC51.15(B3) IC52.2(B2) IC52.6(B1) IC52.11(B4) IC52.15(B3) IC53.2(B2) IC53.6(B1) IC53.11(B4) IC53.12(A4) IC53.14(A3) IC53.15(B3) IC56.1(1G) IC56.6(1C0) IC56.15(2G) IC118.8(A7) IC118.9(A8) IC139.9(G1) IC139.10(G2) IC147.5(EI) IC153.17(B:A4) IC154.11(B:A1) IC154.13(B:A2) IC154.15(B:A3) IC154.17(B:A4) IC196.11(B:A1) IC196.13(B:A2) IC196.15(B:A3) IC196.17(B:A4) IC199.13(A:I4) S1.2(P) S2.3(S) U$1.1(A14) U$1.14(GND) U$1.20(/CE) U$1.22(/OE) U$1.27(/WE) U$2.1(A14) U$2.14(GND) U$2.20(/CE) U$2.22(/OE) U$2.27(/WE) U$3.1(A14) U$3.14(GND) U$3.20(/CE) U$3.22(/OE) U$3.27(/WE) U$4.1(A14) U$4.14(GND) U$4.20(/CE) U$4.22(/OE) U$4.27(/WE) U$5.1(A14) U$5.14(GND) U$5.20(/CE) U$5.22(/OE) U$5.27(/WE) U$6.1(A14) U$6.14(GND) U$6.20(/CE) U$6.22(/OE) U$6.27(/WE) U$7.1(A14) U$7.14(GND) U$7.20(/CE) U$7.22(/OE) U$7.27(/WE) U$8.1(A14) U$8.14(GND) U$8.20(/CE) U$8.22(/OE) U$8.27(/WE) U$9.1(A14) U$9.14(GND) U$9.20(/CE) U$9.22(/OE) U$9.27(/WE)
INT_ENABLE: IC55.13(A:I2) IC190.2(1Q) IC191.11(B:A1)
INT_PENDING: IC55.12(A:O)
INT_STATUS_CODE_OUT: IC153.19(B:G) IC154.19(B:G)
INTERRUPT_STATUS_OUT: IC127.19(B:G) IC152.19(B:G)
MASK_4.5: IC148.12(D:I0)
MASK_5.5: IC49.12(D:I0)
MASK_6.5: IC149.12(D:I0)
MASK_7.5: IC149.9(C:I0)
MASK_ENABLE: IC49.13(D:I1) IC148.13(D:I1) IC149.10(C:I1) IC149.13(D:I1)
MASK_FLAGS_OUT: IC193.19(B:G) IC194.19(B:G)
MASK_FLAGS_WRT: IC128.1(G)
MDR_IN_BUS0: IC21.3(D1)
MDR_IN_BUS1: IC21.4(D2)
MDR_IN_BUS2: IC21.7(D3)
MDR_IN_BUS3: IC21.8(D4)
MDR_IN_BUS4: IC21.13(D5)
MDR_IN_BUS5: IC21.14(D6)
MDR_IN_BUS6: IC21.17(D7)
MDR_IN_BUS7: IC21.18(D8)
MEM/IO: IC10.15(B:A3) IC76.2(Q1)
N$1: IC9.2(A:A1) IC100.2(Q1)
N$2: IC9.4(A:A2) IC100.5(Q2)
N$3: IC9.6(A:A3) IC100.6(Q3)
N$4: IC9.8(A:A4) IC100.9(Q4)
N$5: IC9.11(B:A1) IC100.12(Q5)
N$6: IC9.13(B:A2) IC100.15(Q6)
N$7: IC9.15(B:A3) IC100.16(Q7)
N$8: IC9.17(B:A4) IC100.19(Q8)
N$9: IC9.1(A:G) IC9.19(B:G)
N$10: IC80.6(B:O) IC133.2(A:I1)
N$11: IC111.19(B:G) IC112.19(B:G)
N$12: IC109.19(B:G) IC110.19(B:G)
N$13: IC1.2(Q1) IC2.11(B:A1)
N$14: IC7.2(Q1) IC27.11(B:A1) IC28.11(B:A1)
N$15: IC1.5(Q2) IC2.13(B:A2)
N$16: IC1.6(Q3) IC2.15(B:A3)
N$17: IC1.9(Q4) IC2.17(B:A4)
N$18: IC1.12(Q5) IC3.11(B:A1)
N$19: IC1.15(Q6) IC3.13(B:A2)
N$20: IC1.16(Q7) IC3.15(B:A3)
N$21: IC1.19(Q8) IC3.17(B:A4)
N$22: IC2.19(B:G) IC3.19(B:G)
N$23: IC65.2(A:O) IC138.2(A:I1)
N$24: IC143.3(A:O) IC170.5(B:I1)
N$25: IC101.2(Q1) IC102.11(B:A1)
N$26: IC101.5(Q2) IC102.13(B:A2)
N$27: IC101.6(Q3) IC102.15(B:A3)
N$28: IC101.9(Q4) IC102.17(B:A4)
N$29: IC101.12(Q5) IC117.11(B:A1)
N$30: IC101.15(Q6) IC117.13(B:A2)
N$31: IC101.16(Q7) IC117.15(B:A3)
N$32: IC101.19(Q8) IC117.17(B:A4)
N$33: IC103.2(Q1) IC105.11(B:A1)
N$34: IC103.5(Q2) IC105.13(B:A2)
N$35: IC103.6(Q3) IC105.15(B:A3)
N$36: IC103.9(Q4) IC105.17(B:A4)
N$37: IC103.12(Q5) IC106.11(B:A1)
N$38: IC103.15(Q6) IC106.13(B:A2)
N$39: IC103.16(Q7) IC106.15(B:A3)
N$40: IC103.19(Q8) IC106.17(B:A4)
N$41: IC104.2(Q1) IC107.11(B:A1)
N$42: IC104.5(Q2) IC107.13(B:A2)
N$43: IC104.6(Q3) IC107.15(B:A3)
N$44: IC104.9(Q4) IC107.17(B:A4)
N$45: IC104.12(Q5) IC108.11(B:A1)
N$46: IC104.15(Q6) IC108.13(B:A2)
N$47: IC104.16(Q7) IC108.15(B:A3)
N$48: IC104.19(Q8) IC108.17(B:A4)
N$49: IC102.19(B:G) IC117.19(B:G)
N$50: IC130.6(B:O) IC141.1(A:I) IC143.2(A:I1)
N$51: IC7.5(Q2) IC27.13(B:A2) IC28.13(B:A2)
N$52: IC7.6(Q3) IC27.15(B:A3) IC28.15(B:A3)
N$53: IC7.9(Q4) IC27.17(B:A4) IC28.17(B:A4)
N$54: IC7.12(Q5) IC26.11(B:A1) IC29.11(B:A1)
N$55: IC7.15(Q6) IC26.13(B:A2) IC29.13(B:A2)
N$56: IC7.16(Q7) IC26.15(B:A3) IC29.15(B:A3)
N$57: IC7.19(Q8) IC26.17(B:A4) IC29.17(B:A4)
N$58: IC8.2(Q1) IC25.11(B:A1) IC70.11(B:A1)
N$59: IC8.5(Q2) IC25.13(B:A2) IC70.13(B:A2)
N$60: IC8.6(Q3) IC25.15(B:A3) IC70.15(B:A3)
N$61: IC8.9(Q4) IC25.17(B:A4) IC70.17(B:A4)
N$62: IC8.12(Q5) IC24.11(B:A1) IC71.11(B:A1)
N$63: IC8.15(Q6) IC24.13(B:A2) IC71.13(B:A2)
N$64: IC8.16(Q7) IC24.15(B:A3) IC71.15(B:A3)
N$65: IC105.19(B:G) IC106.19(B:G)
N$66: IC107.19(B:G) IC108.19(B:G)
N$67: IC5.2(Q1) IC109.11(B:A1)
N$68: IC5.5(Q2) IC109.13(B:A2)
N$69: IC5.6(Q3) IC109.15(B:A3)
N$70: IC5.9(Q4) IC109.17(B:A4)
N$71: IC5.12(Q5) IC110.11(B:A1)
N$72: IC5.15(Q6) IC110.13(B:A2)
N$73: IC8.19(Q8) IC24.17(B:A4) IC71.17(B:A4)
N$74: IC200.2(Q1) IC201.2(A:A1)
N$75: IC200.5(Q2) IC201.4(A:A2)
N$76: IC44.2(A:D)
N$77: IC75.3(D1) U$1.11(I/O0)
N$79: IC73.3(1B) IC142.9(2Y)
N$80: IC45.3(B:I) IC74.6(B:O)
N$81: IC138.1(A:I0) IC141.2(A:O)
N$82: IC138.3(A:O) IC170.4(B:I0)
N$83: IC10.2(A:A1) IC13.2(A:A1) IC21.2(Q1) IC30.2(A:A1)
N$84: IC133.1(A:I0) IC170.6(B:O)
N$85: IC64.6(A:O) IC65.1(A:I)
N$86: IC64.2(A:I1) IC150.2(A:O)
N$87: IC144.2(Q1) IC145.11(B:A1)
N$88: IC64.1(A:I0) IC151.2(A:O)
N$89: IC131.6(A:O) IC132.1(A:I)
N$90: IC132.2(A:O) IC143.1(A:I0)
N$91: IC14.2(A0)
N$92: IC14.23(A1)
N$93: IC14.21(A2)
N$94: IC14.19(A3)
N$95: IC15.2(A0)
N$96: IC15.23(A1)
N$97: IC15.21(A2)
N$98: IC15.19(A3)
N$99: IC14.1(B0)
N$100: IC14.22(B1)
N$101: IC14.20(B2)
N$102: IC14.18(B3)
N$103: IC11.12(A:Y4) IC15.1(B0)
N$104: IC11.14(A:Y3) IC15.22(B1)
N$105: IC11.16(A:Y2) IC15.20(B2)
N$106: IC11.18(A:Y1) IC15.18(B3)
N$107: IC14.16(CN+4) IC15.7(CN)
N$108: IC46.4(2D) IC47.7(2Y)
N$109: IC144.5(Q2) IC145.13(B:A2)
N$110: IC131.5(A:I3) IC157.2(A:O)
N$111: IC144.6(Q3) IC145.15(B:A3)
N$112: IC144.9(Q4) IC145.17(B:A4)
N$113: IC131.1(A:I0) IC158.2(A:O)
N$114: IC88.2(Q1) IC89.2(A:A1)
N$115: IC88.5(Q2) IC89.4(A:A2)
N$116: IC88.6(Q3) IC89.6(A:A3)
N$117: IC88.9(Q4) IC89.8(A:A4)
N$118: IC88.12(Q5) IC90.2(A:A1)
N$119: IC88.15(Q6) IC90.4(A:A2)
N$120: IC88.16(Q7) IC90.6(A:A3)
N$121: IC88.19(Q8) IC90.8(A:A4)
N$122: IC86.2(Q1) IC91.2(A:A1)
N$123: IC86.5(Q2) IC91.4(A:A2)
N$124: IC86.6(Q3) IC91.6(A:A3)
N$125: IC86.9(Q4) IC91.8(A:A4)
N$126: IC86.12(Q5) IC92.2(A:A1)
N$127: IC86.15(Q6) IC92.4(A:A2)
N$128: IC86.16(Q7) IC92.6(A:A3)
N$129: IC86.19(Q8) IC92.8(A:A4)
N$130: IC89.1(A:G) IC90.1(A:G)
N$131: IC19.1(A:G) IC19.19(B:G)
N$132: IC10.4(A:A2) IC13.4(A:A2) IC21.5(Q2) IC30.4(A:A2)
N$133: IC91.1(A:G) IC92.1(A:G)
N$134: IC10.6(A:A3) IC13.6(A:A3) IC21.6(Q3) IC30.6(A:A3)
N$135: IC144.12(Q5) IC146.11(B:A1)
N$136: IC144.15(Q6) IC146.13(B:A2)
N$137: IC10.8(A:A4) IC13.8(A:A4) IC21.9(Q4) IC30.8(A:A4)
N$138: IC11.2(A:A1) IC12.2(A:A1) IC21.12(Q5) IC31.2(A:A1)
N$139: IC144.16(Q7) IC146.15(B:A3)
N$140: IC11.4(A:A2) IC12.4(A:A2) IC21.15(Q6) IC31.4(A:A2)
N$141: IC11.6(A:A3) IC12.6(A:A3) IC21.16(Q7) IC31.6(A:A3)
N$142: IC144.19(Q8) IC146.17(B:A4)
N$143: IC5.16(Q7) IC110.15(B:A3)
N$144: IC121.2(Q1) IC122.2(A:A1)
N$145: IC121.5(Q2) IC122.4(A:A2)
N$146: IC5.19(Q8) IC110.17(B:A4)
N$147: IC121.6(Q3) IC122.6(A:A3)
N$148: IC121.9(Q4) IC122.8(A:A4)
N$149: IC121.12(Q5) IC123.2(A:A1)
N$150: IC121.15(Q6) IC123.4(A:A2)
N$151: IC6.2(Q1) IC111.11(B:A1)
N$152: IC121.16(Q7) IC123.6(A:A3)
N$153: IC121.19(Q8) IC123.8(A:A4)
N$154: IC120.2(Q1) IC124.2(A:A1)
N$155: IC120.5(Q2) IC124.4(A:A2)
N$156: IC120.6(Q3) IC124.6(A:A3)
N$157: IC120.9(Q4) IC124.8(A:A4)
N$158: IC120.12(Q5) IC125.2(A:A1)
N$159: IC120.15(Q6) IC125.4(A:A2)
N$160: IC120.16(Q7) IC125.6(A:A3)
N$161: IC120.19(Q8) IC125.8(A:A4)
N$162: IC122.1(A:G) IC123.1(A:G)
N$163: IC124.1(A:G) IC125.1(A:G)
N$164: IC11.8(A:A4) IC12.8(A:A4) IC21.19(Q8) IC31.8(A:A4)
N$165: IC12.1(A:G) IC13.1(A:G)
N$166: IC10.1(A:G) IC11.1(A:G)
N$167: SW3.2
N$168: IC145.19(B:G) IC146.19(B:G)
N$169: IC10.18(A:Y1)
N$170: IC10.16(A:Y2)
N$171: IC10.14(A:Y3)
N$172: IC10.12(A:Y4)
N$175: IC47.5(2A) IC58.3(A:O)
N$176: IC14.7(CN) IC56.7(1Y)
N$177: IC13.18(A:Y1)
N$178: IC13.16(A:Y2)
N$179: IC13.14(A:Y3)
N$180: IC13.12(A:Y4)
N$181: IC12.18(A:Y1)
N$182: IC12.16(A:Y2)
N$183: IC12.14(A:Y3)
N$184: IC12.12(A:Y4)
N$185: IC47.2(1A) IC199.5(A:O)
N$188: IC147.2 IC179.3(A:O)
N$189: IC147.1 IC174.3(A:O)
N$191: IC22.7(2Y)
N$192: IC22.9(3Y)
N$193: IC22.12(4Y)
N$194: IC23.4(1Y)
N$195: IC23.7(2Y)
N$196: IC23.9(3Y)
N$197: IC23.12(4Y)
N$198: IC22.3(1B)
N$199: IC22.6(2B)
N$200: IC30.18(A:Y1)
N$201: IC30.16(A:Y2)
N$202: IC22.1(!A!/B) IC23.1(!A!/B)
N$203: IC30.14(A:Y3)
N$204: IC30.12(A:Y4)
N$205: IC30.1(A:G) IC31.1(A:G)
N$206: IC31.18(A:Y1)
N$207: IC31.16(A:Y2)
N$208: IC31.14(A:Y3)
N$209: IC31.12(A:Y4)
N$210: IC22.4(1Y)
N$211: IC22.10(3B)
N$212: IC22.13(4B)
N$213: IC23.3(1B)
N$214: IC23.6(2B)
N$215: IC23.10(3B)
N$216: IC23.13(4B)
N$217: IC94.2(Q1) IC95.2(A:A1)
N$218: IC46.7(3D) IC47.9(3Y)
N$219: IC46.8(4D) IC47.12(4Y)
N$220: IC147.9(A0) IC153.11(B:A1) IC222.1(A)
N$221: IC147.4 IC155.4(B:O)
N$224: IC149.8(C:O) IC167.1(A:I0)
N$225: IC147.7(A1) IC153.13(B:A2) IC222.2(B)
N$226: IC147.6(A2) IC153.15(B:A3) IC222.3(C)
N$229: IC149.11(D:O) IC174.1(A:I0)
N$230: IC159.4(D2) IC169.5(A:Q)
N$231: IC159.7(D3) IC161.5(A:Q)
N$234: IC49.11(D:O) IC179.1(A:I0)
N$236: IC147.13 IC167.3(A:O)
N$237: IC159.8(D4) IC162.5(A:Q)
N$238: IC159.13(D5) IC163.5(A:Q)
N$239: IC32.3(D1) IC41.7(1Y)
N$240: IC32.11(CLK) IC33.11(CLK)
N$241: IC32.1(CLR) IC33.1(CLR)
N$242: IC32.4(D2) IC41.9(2Y)
N$243: IC32.7(D3) IC40.7(1Y)
N$244: IC32.8(D4) IC40.9(2Y)
N$245: IC32.13(D5) IC34.7(1Y)
N$246: IC32.14(D6) IC34.9(2Y)
N$247: IC33.3(D1) IC35.7(1Y)
N$248: IC33.4(D2) IC35.9(2Y)
N$249: IC147.14(GS) IC183.3(B:I)
N$250: IC33.7(D3) IC36.7(1Y)
N$251: U$2.10(A0)
N$252: U$2.9(A1)
N$253: U$2.8(A2)
N$254: U$2.7(A3)
N$255: U$2.6(A4)
N$256: U$2.5(A5)
N$257: U$2.4(A6)
N$258: U$2.3(A7)
N$259: U$2.25(A8)
N$260: U$2.24(A9)
N$261: U$2.21(A10)
N$262: U$2.23(A11)
N$263: U$2.2(A12)
N$264: U$2.26(A13)
N$265: U$3.10(A0)
N$266: U$3.9(A1)
N$267: U$3.8(A2)
N$268: U$3.7(A3)
N$269: U$3.6(A4)
N$270: U$3.5(A5)
N$271: U$3.4(A6)
N$272: U$3.3(A7)
N$273: U$3.25(A8)
N$274: U$3.24(A9)
N$275: U$3.21(A10)
N$276: U$3.23(A11)
N$277: U$3.2(A12)
N$278: U$3.26(A13)
N$279: U$4.10(A0)
N$280: U$4.9(A1)
N$281: U$4.8(A2)
N$282: U$4.7(A3)
N$283: U$4.6(A4)
N$284: U$4.5(A5)
N$285: U$4.4(A6)
N$286: U$4.3(A7)
N$287: U$4.25(A8)
N$288: U$4.24(A9)
N$289: U$4.21(A10)
N$290: U$4.23(A11)
N$291: U$4.2(A12)
N$292: U$4.26(A13)
N$293: U$5.10(A0)
N$294: U$5.9(A1)
N$295: U$5.8(A2)
N$296: U$5.7(A3)
N$297: U$5.6(A4)
N$298: U$5.5(A5)
N$299: U$5.4(A6)
N$300: U$5.3(A7)
N$301: U$5.25(A8)
N$302: U$5.24(A9)
N$303: U$5.21(A10)
N$304: U$5.23(A11)
N$305: U$5.2(A12)
N$306: U$5.26(A13)
N$307: IC33.8(D4) IC36.9(2Y)
N$308: IC33.13(D5) IC37.7(1Y)
N$309: IC33.14(D6) IC37.9(2Y)
N$310: IC33.17(D7) IC38.7(1Y)
N$311: IC33.18(D8) IC38.9(2Y)
N$312: IC55.2(A:I1) IC147.15(EO)
N$313: IC55.1(A:I0) IC183.4(B:O)
N$315: IC169.1(A:CLR) IC222.14(Y1)
N$316: IC159.14(D6) IC168.5(A:Q)
N$317: IC159.17(D7) IC175.5(A:Q)
N$320: IC20.2(Q1) IC35.4(1C2)
N$321: IC94.5(Q2) IC95.4(A:A2)
N$322: IC148.11(D:O) IC185.1(A:I0)
N$323: IC94.6(Q3) IC95.6(A:A3)
N$324: IC159.18(D8) IC221.5(A:Q)
N$325: IC161.1(A:CLR) IC222.13(Y2)
N$326: IC20.5(Q2) IC35.12(2C2)
N$327: IC20.6(Q3) IC36.4(1C2)
N$328: IC20.9(Q4) IC36.12(2C2)
N$329: IC20.12(Q5) IC37.4(1C2)
N$330: IC20.15(Q6) IC37.12(2C2)
N$331: IC162.1(A:CLR) IC222.12(Y3)
N$332: IC190.9(4Q) IC191.17(B:A4)
N$333: IC50.5(A1)
N$334: IC50.3(A2)
N$335: IC50.14(A3)
N$336: IC50.12(A4)
N$337: IC52.5(A1)
N$338: IC51.5(A1)
N$339: IC51.3(A2)
N$340: IC51.14(A3)
N$341: IC51.12(A4)
N$342: IC20.16(Q7) IC38.4(1C2)
N$343: IC20.19(Q8) IC38.12(2C2)
N$344: IC41.6(1C0) IC50.4(S1)
N$345: IC41.10(2C0) IC50.1(S2)
N$346: IC40.6(1C0) IC50.13(S3)
N$347: IC190.12(5Q) IC192.11(B:A1)
N$348: IC190.15(6Q) IC192.13(B:A2)
N$349: IC40.10(2C0) IC50.10(S4)
N$350: IC52.3(A2)
N$351: IC52.14(A3)
N$352: IC52.12(A4)
N$353: IC53.5(A1)
N$354: IC53.3(A2)
N$355: IC94.9(Q4) IC95.8(A:A4)
N$356: IC94.12(Q5) IC96.2(A:A1)
N$357: IC50.9(C4) IC51.7(C0)
N$358: IC51.9(C4) IC52.7(C0)
N$359: IC52.9(C4) IC53.7(C0)
N$360: IC76.5(Q2)
N$361: IC34.6(1C0) IC51.4(S1)
N$362: IC34.10(2C0) IC51.1(S2)
N$363: IC35.6(1C0) IC51.13(S3)
N$364: IC76.6(Q3)
N$365: IC190.16(7Q) IC192.15(B:A3)
N$366: IC35.10(2C0) IC51.10(S4)
N$367: IC75.4(D2) U$1.12(I/O1)
N$368: IC190.19(8Q) IC192.17(B:A4)
N$369: IC75.7(D3) U$1.13(I/O2)
N$370: IC46.3(1D) IC47.4(1Y)
N$371: IC15.16(CN+4) IC58.2(A:I1)
N$372: IC128.2(1Q) IC193.11(B:A1)
N$373: IC56.3(1C3) IC57.2(A:O)
N$374: IC128.5(2Q) IC193.13(B:A2)
N$375: IC75.8(D4) U$1.15(I/O3)
N$376: IC75.13(D5) U$1.16(I/O4)
N$377: IC75.14(D6) U$1.17(I/O5)
N$378: IC60.3(D1) U$10.11(I/O0)
N$379: IC60.4(D2) U$10.12(I/O1)
N$380: IC60.7(D3) U$10.13(I/O2)
N$381: IC60.8(D4) U$10.15(I/O3)
N$382: IC60.13(D5) U$10.16(I/O4)
N$383: IC60.14(D6) U$10.17(I/O5)
N$384: IC60.17(D7) U$10.18(I/O6)
N$385: IC60.18(D8) U$10.19(I/O7)
N$386: IC61.3(D1) U$11.11(I/O0)
N$387: IC61.4(D2) U$11.12(I/O1)
N$388: IC128.6(3Q) IC193.15(B:A3)
N$389: IC128.9(4Q) IC193.17(B:A4)
N$390: IC128.12(5Q) IC194.11(B:A1)
N$391: IC76.9(Q4)
N$392: IC128.15(6Q) IC194.13(B:A2)
N$393: IC39.2(A:I1) IC43.4(B:O)
N$394: IC39.3(A:O) IC66.1(A:I0)
N$395: IC45.4(B:O) IC66.2(A:I1)
N$396: IC42.4(B:O) IC68.2(A:I1)
N$397: IC66.3(A:O) IC67.4(B:I0)
N$398: IC67.5(B:I1) IC68.3(A:O)
N$399: IC36.6(1C0) IC52.4(S1)
N$400: IC76.12(Q5)
N$401: IC76.15(Q6)
N$402: IC76.16(Q7)
N$403: IC94.15(Q6) IC96.4(A:A2)
N$404: IC6.5(Q2) IC111.13(B:A2)
N$405: IC94.16(Q7) IC96.6(A:A3)
N$406: IC36.10(2C0) IC52.1(S2)
N$407: IC94.19(Q8) IC96.8(A:A4)
N$408: IC93.2(Q1) IC97.2(A:A1)
N$409: IC37.6(1C0) IC52.13(S3)
N$410: IC37.10(2C0) IC52.10(S4)
N$411: IC38.6(1C0) IC53.4(S1)
N$412: IC53.1(S2)
N$413: IC93.5(Q2) IC97.4(A:A2)
N$414: IC93.6(Q3) IC97.6(A:A3)
N$415: IC93.9(Q4) IC97.8(A:A4)
N$416: IC93.12(Q5) IC119.2(A:A1)
N$417: IC93.15(Q6) IC119.4(A:A2)
N$418: IC93.16(Q7) IC119.6(A:A3)
N$419: IC128.16(7Q) IC194.15(B:A3)
N$420: IC93.19(Q8) IC119.8(A:A4)
N$421: IC128.19(8Q) IC194.17(B:A4)
N$422: IC95.1(A:G) IC96.1(A:G)
N$423: IC97.1(A:G) IC119.1(A:G)
N$424: IC17.2(Q1) IC82.2(A:A1)
N$425: IC17.5(Q2) IC82.4(A:A2)
N$426: IC17.6(Q3) IC82.6(A:A3)
N$427: IC17.9(Q4) IC82.8(A:A4)
N$428: IC17.12(Q5) IC83.2(A:A1)
N$429: IC17.15(Q6) IC83.4(A:A2)
N$430: IC17.16(Q7) IC83.6(A:A3)
N$431: IC17.19(Q8) IC83.8(A:A4)
N$432: IC16.2(Q1) IC84.2(A:A1)
N$433: IC16.5(Q2) IC84.4(A:A2)
N$434: IC16.6(Q3) IC84.6(A:A3)
N$435: IC16.9(Q4) IC84.8(A:A4)
N$436: IC16.12(Q5) IC85.2(A:A1)
N$437: IC16.15(Q6) IC85.4(A:A2)
N$438: IC16.16(Q7) IC85.6(A:A3)
N$439: IC16.19(Q8) IC85.8(A:A4)
N$440: IC76.19(Q8)
N$441: IC82.1(A:G) IC83.1(A:G)
N$442: IC76.3(D1) U$2.11(I/O0)
N$443: IC76.4(D2) U$2.12(I/O1)
N$444: IC84.1(A:G) IC85.1(A:G)
N$445: IC77.2(Q1)
N$446: IC197.5(A:O) IC198.1(A:I)
N$447: IC77.5(Q2)
N$448: IC61.7(D3) U$11.13(I/O2)
N$449: IC75.17(D7) U$1.18(I/O6)
N$450: IC75.18(D8) U$1.19(I/O7)
N$451: IC76.7(D3) U$2.13(I/O2)
N$452: IC76.8(D4) U$2.15(I/O3)
N$453: IC76.13(D5) U$2.16(I/O4)
N$454: IC76.14(D6) U$2.17(I/O5)
N$455: IC76.17(D7) U$2.18(I/O6)
N$456: IC76.18(D8) U$2.19(I/O7)
N$457: IC77.3(D1) U$3.11(I/O0)
N$458: IC77.4(D2) U$3.12(I/O1)
N$459: IC77.7(D3) U$3.13(I/O2)
N$460: IC77.8(D4) U$3.15(I/O3)
N$461: IC77.13(D5) U$3.16(I/O4)
N$462: IC77.14(D6) U$3.17(I/O5)
N$463: IC77.17(D7) U$3.18(I/O6)
N$464: IC77.18(D8) U$3.19(I/O7)
N$465: IC78.3(D1) U$4.11(I/O0)
N$466: IC78.4(D2) U$4.12(I/O1)
N$467: IC78.7(D3) U$4.13(I/O2)
N$468: IC78.8(D4) U$4.15(I/O3)
N$469: IC78.13(D5) U$4.16(I/O4)
N$470: IC78.14(D6) U$4.17(I/O5)
N$471: IC78.17(D7) U$4.18(I/O6)
N$472: IC78.18(D8) U$4.19(I/O7)
N$473: IC79.3(D1) U$5.11(I/O0)
N$474: IC79.4(D2) U$5.12(I/O1)
N$475: IC79.7(D3) U$5.13(I/O2)
N$476: IC79.8(D4) U$5.15(I/O3)
N$477: IC79.13(D5) U$5.16(I/O4)
N$478: IC79.14(D6) U$5.17(I/O5)
N$479: IC79.17(D7) U$5.18(I/O6)
N$480: IC79.18(D8) U$5.19(I/O7)
N$481: IC198.2(A:O) IC199.1(A:I0)
N$482: IC61.8(D4) U$11.15(I/O3)
N$483: IC61.13(D5) U$11.16(I/O4)
N$484: IC61.14(D6) U$11.17(I/O5)
N$485: IC61.17(D7) U$11.18(I/O6)
N$486: IC61.18(D8) U$11.19(I/O7)
N$487: IC62.3(D1) U$12.11(I/O0)
N$488: IC62.4(D2) U$12.12(I/O1)
N$489: IC62.7(D3) U$12.13(I/O2)
N$490: IC62.8(D4) U$12.15(I/O3)
N$491: IC62.13(D5) U$12.16(I/O4)
N$492: IC62.14(D6) U$12.17(I/O5)
N$493: IC62.17(D7) U$12.18(I/O6)
N$494: IC62.18(D8) U$12.19(I/O7)
N$495: IC200.6(Q3) IC201.6(A:A3)
N$496: IC200.9(Q4) IC201.8(A:A4)
N$497: IC200.12(Q5) IC202.2(A:A1)
N$498: IC200.15(Q6) IC202.4(A:A2)
N$499: IC129.1(A:G) IC129.19(B:G)
N$500: IC200.16(Q7) IC202.6(A:A3)
N$501: IC200.19(Q8) IC202.8(A:A4)
N$502: IC63.2(Q1) IC203.2(A:A1)
N$503: IC134.18(D8) U$6.19(I/O7)
N$504: IC134.17(D7) U$6.18(I/O6)
N$505: IC134.14(D6) U$6.17(I/O5)
N$506: IC134.13(D5) U$6.16(I/O4)
N$507: IC134.8(D4) U$6.15(I/O3)
N$508: IC134.7(D3) U$6.13(I/O2)
N$509: IC134.4(D2) U$6.12(I/O1)
N$510: IC134.3(D1) U$6.11(I/O0)
N$511: IC135.3(D1) U$7.11(I/O0)
N$512: IC135.4(D2) U$7.12(I/O1)
N$513: IC135.7(D3) U$7.13(I/O2)
N$514: IC135.8(D4) U$7.15(I/O3)
N$515: IC135.13(D5) U$7.16(I/O4)
N$516: IC135.14(D6) U$7.17(I/O5)
N$517: IC135.17(D7) U$7.18(I/O6)
N$518: IC135.18(D8) U$7.19(I/O7)
N$519: IC136.3(D1) U$8.11(I/O0)
N$520: IC136.4(D2) U$8.12(I/O1)
N$521: IC136.7(D3) U$8.13(I/O2)
N$522: IC136.8(D4) U$8.15(I/O3)
N$523: IC136.13(D5) U$8.16(I/O4)
N$524: IC136.14(D6) U$8.17(I/O5)
N$525: IC136.17(D7) U$8.18(I/O6)
N$526: IC136.18(D8) U$8.19(I/O7)
N$527: IC137.3(D1) U$9.11(I/O0)
N$528: IC87.3(A:S2) R1.1 S1.1(O)
N$529: IC87.1(A:R) R2.1 S1.3(S)
N$530: IC44.3(A:CLK) IC54.3(A:CLK) IC139.7(CLK) SW3.C
N$531: IC87.4(A:Q) SW3.1
N$532: SW3.4
N$533: IC137.4(D2) U$9.12(I/O1)
N$534: IC137.7(D3) U$9.13(I/O2)
N$535: IC137.8(D4) U$9.15(I/O3)
N$536: IC137.13(D5) U$9.16(I/O4)
N$537: IC137.14(D6) U$9.17(I/O5)
N$538: IC137.17(D7) U$9.18(I/O6)
N$539: IC137.18(D8) U$9.19(I/O7)
N$540: IC63.5(Q2) IC203.4(A:A2)
N$541: IC63.6(Q3) IC203.6(A:A3)
N$542: IC63.9(Q4) IC203.8(A:A4)
N$543: IC63.12(Q5) IC204.2(A:A1)
N$544: IC63.15(Q6) IC204.4(A:A2)
N$545: IC63.16(Q7) IC204.6(A:A3)
N$546: IC63.19(Q8) IC204.8(A:A4)
N$547: IC201.1(A:G) IC202.1(A:G)
N$548: IC57.3(B:I) IC139.3(Q1)
N$549: IC203.1(A:G) IC204.1(A:G)
N$550: IC48.2(Q1) IC205.2(A:A1)
N$551: IC48.5(Q2) IC205.4(A:A2)
N$552: IC48.6(Q3) IC205.6(A:A3)
N$553: IC48.9(Q4) IC205.8(A:A4)
N$554: IC48.12(Q5) IC206.2(A:A1)
N$555: IC48.15(Q6) IC206.4(A:A2)
N$556: IC48.16(Q7) IC206.6(A:A3)
N$557: IC48.19(Q8) IC206.8(A:A4)
N$558: IC73.2(1A) IC142.7(1Y)
N$559: IC4.2(Q1) IC207.2(A:A1)
N$560: IC4.5(Q2) IC207.4(A:A2)
N$561: IC4.6(Q3) IC207.6(A:A3)
N$562: IC4.9(Q4) IC207.8(A:A4)
N$563: IC4.12(Q5) IC208.2(A:A1)
N$564: IC77.6(Q3)
N$565: IC4.15(Q6) IC208.4(A:A2)
N$566: IC4.16(Q7) IC208.6(A:A3)
N$567: IC81.6(B:O) IC142.11(2C1)
N$568: IC77.9(Q4)
N$569: IC18.6(B:O) IC142.13(2C3)
N$570: IC4.19(Q8) IC208.8(A:A4)
N$571: IC77.12(Q5)
N$572: IC205.1(A:G) IC206.1(A:G)
N$573: IC207.1(A:G) IC208.1(A:G)
N$574: IC210.2(Q1) IC211.2(A:A1)
N$575: IC210.5(Q2) IC211.4(A:A2)
N$576: IC210.6(Q3) IC211.6(A:A3)
N$577: IC6.6(Q3) IC111.15(B:A3)
N$578: IC6.9(Q4) IC111.17(B:A4)
N$579: IC6.12(Q5) IC112.11(B:A1)
N$580: IC6.15(Q6) IC112.13(B:A2)
N$581: IC6.16(Q7) IC112.15(B:A3)
N$582: IC6.19(Q8) IC112.17(B:A4)
N$583: IC98.2(Q1) IC113.11(B:A1)
N$584: IC98.5(Q2) IC113.13(B:A2)
N$585: IC98.6(Q3) IC113.15(B:A3)
N$586: IC98.9(Q4) IC113.17(B:A4)
N$587: IC98.12(Q5) IC114.11(B:A1)
N$588: IC98.15(Q6) IC114.13(B:A2)
N$589: IC98.16(Q7) IC114.15(B:A3)
N$590: IC98.19(Q8) IC114.17(B:A4)
N$591: IC99.2(Q1) IC115.11(B:A1)
N$592: IC99.5(Q2) IC115.13(B:A2)
N$593: IC99.6(Q3) IC115.15(B:A3)
N$594: IC99.9(Q4) IC115.17(B:A4)
N$595: IC99.12(Q5) IC116.11(B:A1)
N$596: IC99.15(Q6) IC116.13(B:A2)
N$597: IC99.16(Q7) IC116.15(B:A3)
N$598: IC99.19(Q8) IC116.17(B:A4)
N$599: IC113.19(B:G) IC114.19(B:G)
N$600: IC115.19(B:G) IC116.19(B:G)
N$601: IC210.9(Q4) IC211.8(A:A4)
N$602: IC77.15(Q6)
N$603: IC210.12(Q5) IC212.2(A:A1)
N$604: IC210.15(Q6) IC212.4(A:A2)
N$605: IC77.16(Q7)
N$606: IC77.19(Q8)
N$607: IC78.2(Q1)
N$608: IC78.5(Q2)
N$609: IC78.6(Q3)
N$610: IC78.9(Q4)
N$611: IC78.12(Q5)
N$612: IC78.15(Q6)
N$613: IC78.16(Q7)
N$614: IC78.19(Q8)
N$615: IC79.2(Q1)
N$616: IC79.5(Q2)
N$617: IC79.6(Q3)
N$618: IC79.9(Q4)
N$619: IC79.12(Q5)
N$620: IC79.15(Q6)
N$621: IC79.16(Q7)
N$622: IC79.19(Q8)
N$623: IC134.2(Q1)
N$624: IC134.5(Q2)
N$625: IC134.6(Q3)
N$626: IC134.9(Q4)
N$627: IC134.12(Q5)
N$628: IC134.15(Q6)
N$629: IC134.16(Q7)
N$630: IC134.19(Q8)
N$631: IC135.2(Q1)
N$632: IC135.5(Q2)
N$633: IC135.6(Q3)
N$634: IC135.9(Q4)
N$635: IC135.12(Q5)
N$636: IC135.15(Q6)
N$637: IC135.16(Q7)
N$638: IC135.19(Q8)
N$639: IC136.2(Q1)
N$640: IC136.5(Q2)
N$641: IC136.6(Q3)
N$642: IC136.9(Q4)
N$643: IC136.12(Q5)
N$644: IC136.15(Q6)
N$645: IC136.16(Q7)
N$646: IC136.19(Q8)
N$647: IC137.2(Q1)
N$648: IC137.5(Q2)
N$649: IC137.6(Q3)
N$650: IC137.9(Q4)
N$651: IC137.12(Q5)
N$652: IC137.15(Q6)
N$653: IC137.16(Q7)
N$654: IC137.19(Q8)
N$655: IC210.16(Q7) IC212.6(A:A3)
N$656: IC210.19(Q8) IC212.8(A:A4)
N$657: IC209.2(Q1) IC213.2(A:A1)
N$658: IC209.5(Q2) IC213.4(A:A2)
N$659: IC209.6(Q3) IC213.6(A:A3)
N$660: IC209.9(Q4) IC213.8(A:A4)
N$661: IC209.12(Q5) IC214.2(A:A1)
N$662: IC209.15(Q6) IC214.4(A:A2)
N$663: IC209.16(Q7) IC214.6(A:A3)
N$664: IC209.19(Q8) IC214.8(A:A4)
N$665: IC211.1(A:G) IC212.1(A:G)
N$666: IC213.1(A:G) IC214.1(A:G)
N$667: IC216.2(Q1) IC217.2(A:A1)
N$668: IC216.5(Q2) IC217.4(A:A2)
N$669: IC216.6(Q3) IC217.6(A:A3)
N$670: IC216.9(Q4) IC217.8(A:A4)
N$671: IC216.12(Q5) IC218.2(A:A1)
N$672: IC216.15(Q6) IC218.4(A:A2)
N$673: IC216.16(Q7) IC218.6(A:A3)
N$674: IC216.19(Q8) IC218.8(A:A4)
N$675: IC215.2(Q1) IC219.2(A:A1)
N$676: IC215.5(Q2) IC219.4(A:A2)
N$677: IC215.6(Q3) IC219.6(A:A3)
N$678: IC215.9(Q4) IC219.8(A:A4)
N$679: IC215.12(Q5) IC220.2(A:A1)
N$680: IC215.15(Q6) IC220.4(A:A2)
N$681: IC215.16(Q7) IC220.6(A:A3)
N$682: IC215.19(Q8) IC220.8(A:A4)
N$683: IC217.1(A:G) IC218.1(A:G)
N$684: IC219.1(A:G) IC220.1(A:G)
N$685: IC163.1(A:CLR) IC222.11(Y4)
N$686: IC168.1(A:CLR) IC222.10(Y5)
N$687: IC175.1(A:CLR) IC222.9(Y6)
N$688: IC221.1(A:CLR) IC222.7(Y7)
NOT_COND: IC74.4(B:I0)
NOT_RST: IC4.1(CLR) IC5.1(CLR) IC6.1(CLR) IC7.1(CLR) IC8.1(CLR) IC16.1(CLR) IC17.1(CLR) IC20.1(CLR) IC21.1(CLR) IC48.1(CLR) IC63.1(CLR) IC75.1(CLR) IC76.1(CLR) IC77.1(CLR) IC78.1(CLR) IC79.1(CLR) IC86.1(CLR) IC88.1(CLR) IC93.1(CLR) IC94.1(CLR) IC99.1(CLR) IC103.1(CLR) IC104.1(CLR) IC120.1(CLR) IC121.1(CLR) IC134.1(CLR) IC135.1(CLR) IC136.1(CLR) IC137.1(CLR) IC200.1(CLR) IC209.1(CLR) IC210.1(CLR) IC215.1(CLR) IC216.1(CLR)
OF: IC46.9(4Q) IC59.14(4A) IC195.17(B:A4)
OF_FROM_ALU: IC47.14(4A) IC126.8(4D)
RD: IC10.11(B:A1) IC75.16(Q7)
RST: IC54.2(A:D) IC54.5(A:Q) IC139.15(CLR) R3.1 S2.2(P)
RST5.5: IC161.3(A:CLK)
RST6.5: IC162.3(A:CLK)
RST_4.5: IC127.13(B:A2) IC159.5(Q2) IC185.2(A:I1)
RST_5.5: IC127.15(B:A3) IC159.6(Q3) IC179.2(A:I1)
RST_6.5: IC127.17(B:A4) IC159.9(Q4) IC174.2(A:I1)
RST_7.5: IC152.11(B:A1) IC159.12(Q5) IC167.2(A:I1)
RST_8.5: IC147.12 IC152.13(B:A2) IC159.15(Q6)
SF: IC46.6(3Q) IC59.11(3A) IC195.15(B:A3)
SF_FROM_ALU: IC126.7(3D)
SF_XOR_OF: IC72.6(B:O) IC81.4(B:I0) IC142.10(2C0)
STOP_CLK: IC44.5(A:Q) IC139.1(M) IC139.2(N)
TRAP: IC169.3(A:CLK)
TYP_0: IC39.1(A:I0) IC42.3(B:I) IC69.1(A:I0)
TYP_1: IC43.3(B:I) IC68.1(A:I0) IC69.2(A:I1)
U_AD0: IC32.2(Q1) IC140.2(A1) U$6.10(A0) U$7.10(A0) U$8.10(A0) U$9.10(A0)
U_AD1: IC32.5(Q2) IC140.3(A2) U$6.9(A1) U$7.9(A1) U$8.9(A1) U$9.9(A1)
U_AD2: IC32.6(Q3) IC140.4(A3) U$6.8(A2) U$7.8(A2) U$8.8(A2) U$9.8(A2)
U_AD3: IC32.9(Q4) IC140.5(A4) U$6.7(A3) U$7.7(A3) U$8.7(A3) U$9.7(A3)
U_AD4: IC32.12(Q5) IC140.6(A5) U$6.6(A4) U$7.6(A4) U$8.6(A4) U$9.6(A4)
U_AD5: IC32.15(Q6) IC140.7(A6) U$6.5(A5) U$7.5(A5) U$8.5(A5) U$9.5(A5)
U_AD6: IC32.16(Q7) IC140.8(A7) U$6.4(A6) U$7.4(A6) U$8.4(A6) U$9.4(A6)
U_AD7: IC32.19(Q8) IC140.9(A8) U$6.3(A7) U$7.3(A7) U$8.3(A7) U$9.3(A7)
U_AD8: IC33.2(Q1) U$6.25(A8) U$7.25(A8) U$8.25(A8) U$9.25(A8)
U_AD9: IC33.5(Q2) IC118.2(A1) IC118.3(A2) U$6.24(A9) U$7.24(A9) U$8.24(A9) U$9.24(A9)
U_AD10: IC33.6(Q3) IC118.4(A3) U$6.21(A10) U$7.21(A10) U$8.21(A10) U$9.21(A10)
U_AD11: IC33.9(Q4) IC118.5(A4) U$6.23(A11) U$7.23(A11) U$8.23(A11) U$9.23(A11)
U_AD12: IC33.12(Q5) IC118.6(A5) U$6.2(A12) U$7.2(A12) U$8.2(A12) U$9.2(A12)
U_AD13: IC33.15(Q6) IC118.7(A6) U$6.26(A13) U$7.26(A13) U$8.26(A13) U$9.26(A13)
U_AD_BUFF0: IC140.18(Y1) U$1.10(A0)
U_AD_BUFF1: IC140.17(Y2) U$1.9(A1)
U_AD_BUFF2: IC140.16(Y3) U$1.8(A2)
U_AD_BUFF3: IC140.15(Y4) U$1.7(A3)
U_AD_BUFF4: IC140.14(Y5) U$1.6(A4)
U_AD_BUFF5: IC140.13(Y6) U$1.5(A5)
U_AD_BUFF6: IC140.12(Y7) U$1.4(A6)
U_AD_BUFF7: IC140.11(Y8) U$1.3(A7)
U_AD_BUFF8: IC118.18(Y1) U$1.25(A8)
U_AD_BUFF9: IC118.17(Y2) U$1.24(A9)
U_AD_BUFF10: IC118.16(Y3) U$1.21(A10)
U_AD_BUFF11: IC118.15(Y4) U$1.23(A11)
U_AD_BUFF12: IC118.14(Y5) U$1.2(A12)
U_AD_BUFF13: IC118.13(Y6) U$1.26(A13)
U_ADDR_MUX_0: IC34.14(A) IC35.14(A) IC36.14(A) IC37.14(A) IC38.14(A) IC40.14(A) IC41.14(A) IC67.6(B:O)
U_ADDR_MUX_1: IC34.2(B) IC35.2(B) IC36.2(B) IC37.2(B) IC38.2(B) IC40.2(B) IC41.2(B) IC69.3(A:O)
U_CF: IC59.6(2B) IC126.5(2Q)
U_FLAGS_WRT: IC126.1(G)
U_OF: IC59.13(4B) IC126.9(4Q)
U_SF: IC59.10(3B) IC126.6(3Q)
U_ZF: IC59.3(1B) IC126.2(1Q)
VCC: IC50.6(B1) IC56.5(1C1) IC161.2(A:D) IC162.2(A:D) IC163.2(A:D) IC168.2(A:D) IC169.2(A:D) IC175.2(A:D) IC221.2(A:D) IC222.6(G1) R1.2 R2.2 R3.2
WR: IC10.13(B:A2) IC75.19(Q8)
XBUS0: IC2.9(B:Y1) IC9.18(A:Y1) IC25.9(B:Y1) IC27.9(B:Y1) IC95.18(A:Y1) IC97.18(A:Y1) IC102.9(B:Y1) IC105.9(B:Y1) IC107.9(B:Y1) IC109.9(B:Y1) IC111.9(B:Y1) IC113.9(B:Y1) IC115.9(B:Y1) IC122.18(A:Y1) IC124.18(A:Y1) IC127.9(B:Y1) IC129.18(A:Y1) IC153.9(B:Y1) IC191.9(B:Y1) IC193.9(B:Y1) IC195.9(B:Y1)
XBUS1: IC2.7(B:Y2) IC9.16(A:Y2) IC25.7(B:Y2) IC27.7(B:Y2) IC95.16(A:Y2) IC97.16(A:Y2) IC102.7(B:Y2) IC105.7(B:Y2) IC107.7(B:Y2) IC109.7(B:Y2) IC111.7(B:Y2) IC113.7(B:Y2) IC115.7(B:Y2) IC122.16(A:Y2) IC124.16(A:Y2) IC127.7(B:Y2) IC129.16(A:Y2) IC153.7(B:Y2) IC191.7(B:Y2) IC193.7(B:Y2) IC195.7(B:Y2)
XBUS2: IC2.5(B:Y3) IC9.14(A:Y3) IC25.5(B:Y3) IC27.5(B:Y3) IC95.14(A:Y3) IC97.14(A:Y3) IC102.5(B:Y3) IC105.5(B:Y3) IC107.5(B:Y3) IC109.5(B:Y3) IC111.5(B:Y3) IC113.5(B:Y3) IC115.5(B:Y3) IC122.14(A:Y3) IC124.14(A:Y3) IC127.5(B:Y3) IC129.14(A:Y3) IC153.5(B:Y3) IC191.5(B:Y3) IC193.5(B:Y3) IC195.5(B:Y3)
XBUS3: IC2.3(B:Y4) IC9.12(A:Y4) IC25.3(B:Y4) IC27.3(B:Y4) IC95.12(A:Y4) IC97.12(A:Y4) IC102.3(B:Y4) IC105.3(B:Y4) IC107.3(B:Y4) IC109.3(B:Y4) IC111.3(B:Y4) IC113.3(B:Y4) IC115.3(B:Y4) IC122.12(A:Y4) IC124.12(A:Y4) IC127.3(B:Y4) IC129.12(A:Y4) IC153.3(B:Y4) IC191.3(B:Y4) IC193.3(B:Y4) IC195.3(B:Y4)
XBUS4: IC3.9(B:Y1) IC9.9(B:Y1) IC24.9(B:Y1) IC26.9(B:Y1) IC96.18(A:Y1) IC106.9(B:Y1) IC108.9(B:Y1) IC110.9(B:Y1) IC112.9(B:Y1) IC114.9(B:Y1) IC116.9(B:Y1) IC117.9(B:Y1) IC119.18(A:Y1) IC123.18(A:Y1) IC125.18(A:Y1) IC129.9(B:Y1) IC152.9(B:Y1) IC154.9(B:Y1) IC192.9(B:Y1) IC194.9(B:Y1) IC196.9(B:Y1)
XBUS5: IC3.7(B:Y2) IC9.7(B:Y2) IC24.7(B:Y2) IC26.7(B:Y2) IC96.16(A:Y2) IC106.7(B:Y2) IC108.7(B:Y2) IC110.7(B:Y2) IC112.7(B:Y2) IC114.7(B:Y2) IC116.7(B:Y2) IC117.7(B:Y2) IC119.16(A:Y2) IC123.16(A:Y2) IC125.16(A:Y2) IC129.7(B:Y2) IC152.7(B:Y2) IC154.7(B:Y2) IC192.7(B:Y2) IC194.7(B:Y2) IC196.7(B:Y2)
XBUS6: IC3.5(B:Y3) IC9.5(B:Y3) IC24.5(B:Y3) IC26.5(B:Y3) IC96.14(A:Y3) IC106.5(B:Y3) IC108.5(B:Y3) IC110.5(B:Y3) IC112.5(B:Y3) IC114.5(B:Y3) IC116.5(B:Y3) IC117.5(B:Y3) IC119.14(A:Y3) IC123.14(A:Y3) IC125.14(A:Y3) IC129.5(B:Y3) IC152.5(B:Y3) IC154.5(B:Y3) IC192.5(B:Y3) IC194.5(B:Y3) IC196.5(B:Y3)
XBUS7: IC3.3(B:Y4) IC9.3(B:Y4) IC24.3(B:Y4) IC26.3(B:Y4) IC80.4(B:I0) IC96.12(A:Y4) IC106.3(B:Y4) IC108.3(B:Y4) IC110.3(B:Y4) IC112.3(B:Y4) IC114.3(B:Y4) IC116.3(B:Y4) IC117.3(B:Y4) IC119.12(A:Y4) IC123.12(A:Y4) IC125.12(A:Y4) IC129.3(B:Y4) IC130.5(B:I1) IC152.3(B:Y4) IC154.3(B:Y4) IC192.3(B:Y4) IC194.3(B:Y4) IC196.3(B:Y4)
XBUS8: IC145.9(B:Y1)
XBUS9: IC145.7(B:Y2)
XBUS10: IC145.5(B:Y3)
XBUS11: IC145.3(B:Y4)
XBUS12: IC146.9(B:Y1)
XBUS13: IC146.7(B:Y2)
XBUS14: IC146.5(B:Y3)
XBUS15: IC146.3(B:Y4)
XBUS16: IC82.18(A:Y1) IC84.18(A:Y1) IC89.18(A:Y1) IC91.18(A:Y1)
XBUS17: IC82.16(A:Y2) IC84.16(A:Y2) IC89.16(A:Y2) IC91.16(A:Y2)
XBUS18: IC82.14(A:Y3) IC84.14(A:Y3) IC89.14(A:Y3) IC91.14(A:Y3)
XBUS19: IC82.12(A:Y4) IC84.12(A:Y4) IC89.12(A:Y4) IC91.12(A:Y4)
XBUS20: IC83.18(A:Y1) IC85.18(A:Y1) IC90.18(A:Y1) IC92.18(A:Y1)
XBUS21: IC83.16(A:Y2) IC85.16(A:Y2) IC90.16(A:Y2) IC92.16(A:Y2)
XBUS22: IC83.14(A:Y3) IC85.14(A:Y3) IC90.14(A:Y3) IC92.14(A:Y3)
XBUS23: IC83.12(A:Y4) IC85.12(A:Y4) IC90.12(A:Y4) IC92.12(A:Y4)
XBUS24: IC217.18(A:Y1) IC219.18(A:Y1)
XBUS25: IC217.16(A:Y2) IC219.16(A:Y2)
XBUS26: IC217.14(A:Y3) IC219.14(A:Y3)
XBUS27: IC217.12(A:Y4) IC219.12(A:Y4)
XBUS28: IC218.18(A:Y1) IC220.18(A:Y1)
XBUS29: IC218.16(A:Y2) IC220.16(A:Y2)
XBUS30: IC218.14(A:Y3) IC220.14(A:Y3)
XBUS31: IC218.12(A:Y4) IC220.12(A:Y4)
YBUS0: IC19.18(A:Y1)
YBUS1: IC19.16(A:Y2)
YBUS2: IC19.14(A:Y3)
YBUS3: IC19.12(A:Y4)
YBUS4: IC19.9(B:Y1)
YBUS5: IC19.7(B:Y2)
YBUS6: IC19.5(B:Y3)
YBUS7: IC19.3(B:Y4) IC130.4(B:I0)
YBUS8: IC201.18(A:Y1) IC203.18(A:Y1) IC205.18(A:Y1) IC207.18(A:Y1)
YBUS9: IC201.16(A:Y2) IC203.16(A:Y2) IC205.16(A:Y2) IC207.16(A:Y2)
YBUS10: IC201.14(A:Y3) IC203.14(A:Y3) IC205.14(A:Y3) IC207.14(A:Y3)
YBUS11: IC201.12(A:Y4) IC205.12(A:Y4) IC207.12(A:Y4)
YBUS12: IC202.18(A:Y1) IC204.18(A:Y1) IC206.18(A:Y1) IC208.18(A:Y1)
YBUS13: IC202.16(A:Y2) IC204.16(A:Y2) IC206.16(A:Y2) IC208.16(A:Y2)
YBUS14: IC202.14(A:Y3) IC204.14(A:Y3) IC206.14(A:Y3) IC208.14(A:Y3)
YBUS15: IC202.12(A:Y4) IC204.12(A:Y4) IC206.12(A:Y4) IC208.12(A:Y4)
YBUS16: IC211.18(A:Y1) IC213.18(A:Y1)
YBUS17: IC211.16(A:Y2) IC213.16(A:Y2)
YBUS18: IC211.14(A:Y3) IC213.14(A:Y3)
YBUS19: IC211.12(A:Y4) IC213.12(A:Y4)
YBUS20: IC212.18(A:Y1) IC214.18(A:Y1)
YBUS21: IC212.16(A:Y2) IC214.16(A:Y2)
YBUS22: IC212.14(A:Y3) IC214.14(A:Y3)
YBUS23: IC212.12(A:Y4) IC214.12(A:Y4)
ZBUFF0_0: IC93.3(D1) IC94.3(D1) IC120.3(D1) IC121.3(D1)
ZBUFF0_1: IC93.4(D2) IC94.4(D2) IC120.4(D2) IC121.4(D2)
ZBUFF0_2: IC93.7(D3) IC94.7(D3) IC120.7(D3) IC121.7(D3)
ZBUFF0_3: IC93.8(D4) IC94.8(D4) IC120.8(D4) IC121.8(D4)
ZBUFF0_4: IC93.13(D5) IC94.13(D5) IC120.13(D5) IC121.13(D5)
ZBUFF0_5: IC93.14(D6) IC94.14(D6) IC120.14(D6)
ZBUFF0_6: IC93.17(D7) IC94.17(D7) IC120.17(D7) IC121.14(D6) IC121.17(D7)
ZBUFF0_7: IC93.18(D8) IC94.18(D8) IC120.18(D8) IC121.18(D8)
ZBUFF0_8: IC4.3(D1) IC48.3(D1) IC63.3(D1) IC200.3(D1)
ZBUFF0_9: IC4.4(D2) IC48.4(D2) IC63.4(D2) IC200.4(D2)
ZBUFF0_10: IC4.7(D3) IC48.7(D3) IC63.7(D3) IC200.7(D3)
ZBUFF0_11: IC4.8(D4) IC48.8(D4) IC63.8(D4) IC200.8(D4)
ZBUFF0_12: IC4.13(D5) IC48.13(D5) IC63.13(D5) IC200.13(D5)
ZBUFF0_13: IC4.14(D6) IC48.14(D6) IC63.14(D6) IC200.14(D6)
ZBUFF0_14: IC4.17(D7) IC48.17(D7) IC63.17(D7) IC200.17(D7)
ZBUFF0_15: IC4.18(D8) IC48.18(D8) IC63.18(D8) IC200.18(D8)
ZBUFF0_16: IC16.3(D1) IC17.3(D1) IC86.3(D1) IC88.3(D1)
ZBUFF0_17: IC16.4(D2) IC17.4(D2) IC86.4(D2) IC88.4(D2)
ZBUFF0_18: IC16.7(D3) IC17.7(D3) IC86.7(D3) IC88.7(D3)
ZBUFF0_19: IC16.8(D4) IC17.8(D4) IC86.8(D4) IC88.8(D4)
ZBUFF0_20: IC16.13(D5) IC17.13(D5) IC86.13(D5) IC88.13(D5)
ZBUFF0_21: IC16.14(D6) IC17.14(D6) IC86.14(D6)
ZBUFF0_22: IC16.17(D7) IC17.17(D7) IC86.17(D7) IC88.14(D6) IC88.17(D7)
ZBUFF0_23: IC16.18(D8) IC17.18(D8) IC86.18(D8) IC88.18(D8)
ZBUFF0_24: IC209.3(D1) IC210.3(D1)
ZBUFF0_25: IC209.4(D2) IC210.4(D2)
ZBUFF0_26: IC209.7(D3) IC210.7(D3)
ZBUFF0_27: IC209.8(D4) IC210.8(D4)
ZBUFF0_28: IC209.13(D5) IC210.13(D5)
ZBUFF0_29: IC209.14(D6) IC210.14(D6)
ZBUFF0_30: IC209.17(D7) IC210.17(D7)
ZBUFF0_31: IC209.18(D8) IC210.18(D8)
ZBUFF0_32: IC215.3(D1) IC216.3(D1)
ZBUFF0_33: IC215.4(D2) IC216.4(D2)
ZBUFF0_34: IC215.7(D3) IC216.7(D3)
ZBUFF0_35: IC215.8(D4) IC216.8(D4)
ZBUFF0_36: IC215.13(D5) IC216.13(D5)
ZBUFF0_37: IC215.14(D6) IC216.14(D6)
ZBUFF0_38: IC215.17(D7) IC216.17(D7)
ZBUFF0_39: IC215.18(D8) IC216.18(D8)
ZBUFF1_0: IC5.3(D1) IC6.3(D1) IC7.3(D1) IC8.3(D1) IC98.3(D1) IC99.3(D1) IC103.3(D1) IC104.3(D1)
ZBUFF1_1: IC5.4(D2) IC6.4(D2) IC7.4(D2) IC8.4(D2) IC98.4(D2) IC99.4(D2) IC103.4(D2) IC104.4(D2)
ZBUFF1_2: IC5.7(D3) IC6.7(D3) IC7.7(D3) IC8.7(D3) IC98.7(D3) IC99.7(D3) IC103.7(D3) IC104.7(D3)
ZBUFF1_3: IC5.8(D4) IC6.8(D4) IC7.8(D4) IC8.8(D4) IC98.8(D4) IC99.8(D4) IC103.8(D4) IC104.8(D4)
ZBUFF1_4: IC5.13(D5) IC6.13(D5) IC7.13(D5) IC8.13(D5) IC98.13(D5) IC99.13(D5) IC103.13(D5) IC104.13(D5)
ZBUFF1_5: IC5.14(D6) IC6.14(D6) IC7.14(D6) IC8.14(D6) IC98.14(D6) IC99.14(D6) IC103.14(D6) IC104.14(D6)
ZBUFF1_6: IC5.17(D7) IC6.17(D7) IC7.17(D7) IC8.17(D7) IC98.17(D7) IC99.17(D7) IC103.17(D7) IC104.17(D7)
ZBUFF1_7: IC5.18(D8) IC6.18(D8) IC7.18(D8) IC8.18(D8) IC98.18(D8) IC99.18(D8) IC103.18(D8) IC104.18(D8)
ZBUFF2_0: IC1.3(D1) IC23.14(4A) IC47.3(1B) IC100.3(D1) IC101.3(D1)
ZBUFF2_1: IC1.4(D2) IC23.11(3A) IC47.6(2B) IC100.4(D2) IC101.4(D2)
ZBUFF2_2: IC1.7(D3) IC23.5(2A) IC47.10(3B) IC100.7(D3) IC101.7(D3)
ZBUFF2_3: IC1.8(D4) IC23.2(1A) IC47.13(4B) IC100.8(D4) IC101.8(D4)
ZBUFF2_4: IC1.13(D5) IC22.14(4A) IC100.13(D5) IC101.13(D5)
ZBUFF2_5: IC1.14(D6) IC22.11(3A) IC100.14(D6) IC101.14(D6)
ZBUFF2_6: IC1.17(D7) IC22.5(2A) IC100.17(D7) IC101.17(D7)
ZBUFF2_7: IC1.18(D8) IC22.2(1A)
ZBUFF2_8: IC144.3(D1)
ZBUFF2_9: IC144.4(D2)
ZBUFF2_10: IC144.7(D3)
ZBUFF2_11: IC144.8(D4)
ZBUFF2_12: IC144.13(D5)
ZBUFF2_13: IC144.14(D6)
ZBUFF2_14: IC144.17(D7)
ZBUS0: IC14.9(F0) IC128.3(1D) IC190.3(1D) IC197.1(A:I0)
ZBUS1: IC14.10(F1) IC128.4(2D) IC190.4(2D) IC197.2(A:I1)
ZBUS2: IC14.11(F2) IC128.7(3D) IC190.7(3D) IC197.3(A:I2)
ZBUS3: IC14.13(F3) IC128.8(4D) IC190.8(4D) IC197.12(A:I3)
ZBUS4: IC15.13(F3) IC128.13(5D) IC190.13(5D) IC197.13(A:I4)
ZBUS5: IC15.11(F2) IC128.14(6D) IC190.14(6D) IC199.2(A:I1)
ZBUS6: IC15.10(F1) IC128.17(7D) IC190.17(7D) IC199.3(A:I2)
ZBUS7: IC15.9(F0) IC47.11(3A) IC80.5(B:I1) IC128.18(8D) IC190.18(8D) IC199.12(A:I3)
ZF: IC46.2(1Q) IC59.2(1A) IC195.11(B:A1)
ZF_FROM_ALU: IC126.3(1D)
